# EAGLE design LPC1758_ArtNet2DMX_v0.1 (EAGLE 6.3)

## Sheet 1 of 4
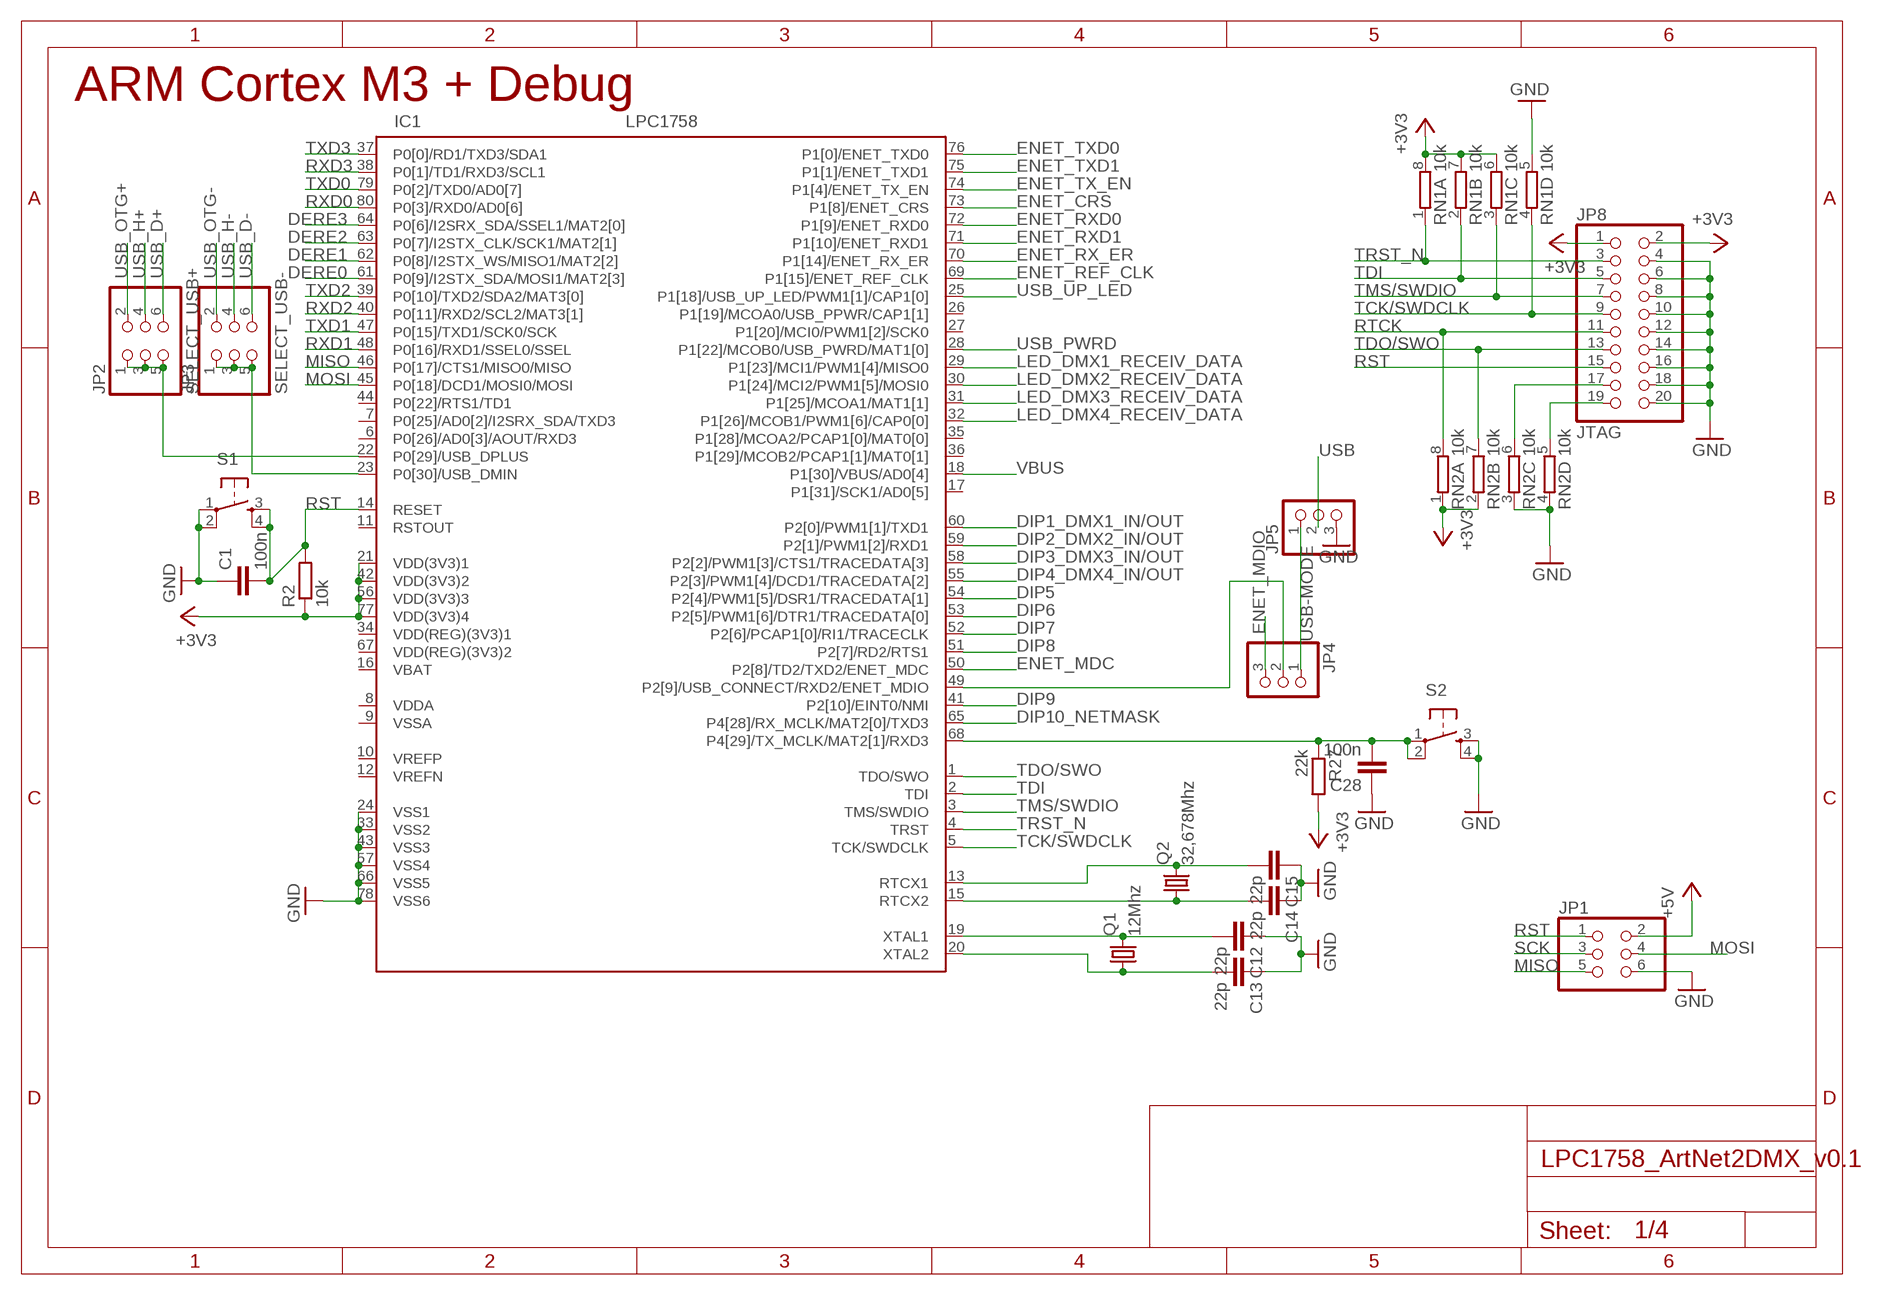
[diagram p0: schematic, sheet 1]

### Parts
C1  100n  C-EUC0805K  [C0805K]
C12  22p  C-EUC0805K  [C0805K]
C13  22p  C-EUC0805K  [C0805K]
C14  22p  C-EUC0805K  [C0805K]
C15  22p  C-EUC0805K  [C0805K]
C28  100n  C-EUC0805K  [C0805K]
IC1  LPC1758  [LQFP80-12X12]
JP1  PINHD-2X3_2.54-SMD  [2X03SMD]
JP2  SELECT_USB+  PINHD-2X3_2.54-SMD  [2X03SMD]
JP3  SELECT_USB-  PINHD-2X3_2.54-SMD  [2X03SMD]
JP4  PINHD-1X3_2.54-SMD  [1X03SMD]
JP5  PINHD-1X3_2.54-SMD  [1X03SMD]
JP8  JTAG  PINHD-2X10_2.54  [2X10]
Q1  12Mhz  CRYSTALSM49  [SM49]
Q2  32,678Mhz  CRYSTALSM49  [SM49]
R2  10k  R-EU_R0805  [R0805]
R27  22k  R-EU_R0805  [R0805]
RN1  10k  4R-NEXBS8V  [EXBS8V]
RN2  10k  4R-NEXBS8V  [EXBS8V]
S1  TASTER_93XX  [TASTER_93XX]
S2  TASTER_93XX  [TASTER_93XX]

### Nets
+3V3: IC1.21(VDD(3V3)1) IC1.42(VDD(3V3)2) IC1.56(VDD(3V3)3) IC1.77(VDD(3V3)4) JP8.1 JP8.2 R2.1 R27.2 RN1.6 RN1.7 RN1.8 RN2.1 RN2.2 ; also sheet 2,3,4
+5V: JP1.2 ; also sheet 3,4
BUTTON_RESERVE: C28.2 IC1.68(P4[29]/TX_MCLK/MAT2[1]/RXD3) R27.1 S2.1(P) S2.2(P1)
DERE0: IC1.61(P0[9]/I2STX_SDA/MOSI1/MAT2[3]) ; also sheet 3
DERE1: IC1.62(P0[8]/I2STX_WS/MISO1/MAT2[2]) ; also sheet 3
DERE2: IC1.63(P0[7]/I2STX_CLK/SCK1/MAT2[1]) ; also sheet 3
DERE3: IC1.64(P0[6]/I2SRX_SDA/SSEL1/MAT2[0]) ; also sheet 3
DIP1_DMX1_IN/OUT: IC1.60(P2[0]/PWM1[1]/TXD1) ; also sheet 3
DIP2_DMX2_IN/OUT: IC1.59(P2[1]/PWM1[2]/RXD1) ; also sheet 3
DIP3_DMX3_IN/OUT: IC1.58(P2[2]/PWM1[3]/CTS1/TRACEDATA[3]) ; also sheet 3
DIP4_DMX4_IN/OUT: IC1.55(P2[3]/PWM1[4]/DCD1/TRACEDATA[2]) ; also sheet 3
DIP5: IC1.54(P2[4]/PWM1[5]/DSR1/TRACEDATA[1]) ; also sheet 3
DIP6: IC1.53(P2[5]/PWM1[6]/DTR1/TRACEDATA[0]) ; also sheet 3
DIP7: IC1.52(P2[6]/PCAP1[0]/RI1/TRACECLK) ; also sheet 3
DIP8: IC1.51(P2[7]/RD2/RTS1) ; also sheet 3
DIP9: IC1.41(P2[10]/EINT0/NMI) ; also sheet 3
DIP10_NETMASK: IC1.65(P4[28]/RX_MCLK/MAT2[0]/TXD3) ; also sheet 3
ENET_CRS: IC1.73(P1[8]/ENET_CRS) ; also sheet 2
ENET_MDC: IC1.50(P2[8]/TD2/TXD2/ENET_MDC) ; also sheet 2
ENET_MDIO: JP4.3 ; also sheet 2
ENET_REF_CLK: IC1.69(P1[15]/ENET_REF_CLK) ; also sheet 2
ENET_RX_ER: IC1.70(P1[14]/ENET_RX_ER) ; also sheet 2
ENET_RXD0: IC1.72(P1[9]/ENET_RXD0) ; also sheet 2
ENET_RXD1: IC1.71(P1[10]/ENET_RXD1) ; also sheet 2
ENET_TX_EN: IC1.74(P1[4]/ENET_TX_EN) ; also sheet 2
ENET_TXD0: IC1.76(P1[0]/ENET_TXD0) ; also sheet 2
ENET_TXD1: IC1.75(P1[1]/ENET_TXD1) ; also sheet 2
GND: C1.1 C12.1 C13.1 C14.1 C15.1 C28.1 IC1.24(VSS1) IC1.33(VSS2) IC1.43(VSS3) IC1.57(VSS4) IC1.66(VSS5) IC1.78(VSS6) JP1.6 JP5.3 JP8.4 JP8.6 JP8.8 JP8.10 JP8.12 JP8.14 JP8.16 JP8.18 JP8.20 RN1.5 RN2.3 RN2.4 S1.1(P) S1.2(P1) S2.3(S) S2.4(S1) ; also sheet 2,3,4
LED_DMX1_RECEIV_DATA: IC1.29(P1[23]/MCI1/PWM1[4]/MISO0) ; also sheet 3
LED_DMX2_RECEIV_DATA: IC1.30(P1[24]/MCI2/PWM1[5]/MOSI0) ; also sheet 3
LED_DMX3_RECEIV_DATA: IC1.31(P1[25]/MCOA1/MAT1[1]) ; also sheet 3
LED_DMX4_RECEIV_DATA: IC1.32(P1[26]/MCOB1/PWM1[6]/CAP0[0]) ; also sheet 3
MISO: IC1.46(P0[17]/CTS1/MISO0/MISO) JP1.5
MOSI: IC1.45(P0[18]/DCD1/MOSI0/MOSI) JP1.4
N$12: C12.2 IC1.19(XTAL1) Q1.2
N$13: C13.2 IC1.20(XTAL2) Q1.1
N$16: C14.2 IC1.15(RTCX2) Q2.1
N$20: C15.2 IC1.13(RTCX1) Q2.2
N$22: IC1.22(P0[29]/USB_DPLUS) JP2.1 JP2.3 JP2.5
N$23: IC1.23(P0[30]/USB_DMIN) JP3.1 JP3.3 JP3.5
N$25: IC1.49(P2[9]/USB_CONNECT/RXD2/ENET_MDIO) JP4.2
N$42: JP8.19 RN2.5
N$43: JP8.17 RN2.6
RST: C1.2 IC1.14(RESET) JP1.1 JP8.15 R2.2 S1.3(S) S1.4(S1) ; also sheet 2
RTCK: JP8.11 RN2.8
RXD0: IC1.80(P0[3]/RXD0/AD0[6]) ; also sheet 3
RXD1: IC1.48(P0[16]/RXD1/SSEL0/SSEL) ; also sheet 3
RXD2: IC1.40(P0[11]/RXD2/SCL2/MAT3[1]) ; also sheet 3
RXD3: IC1.38(P0[1]/TD1/RXD3/SCL1) ; also sheet 3
SCK: JP1.3
TCK/SWDCLK: IC1.5(TCK/SWDCLK) JP8.9 RN1.4
TDI: IC1.2(TDI) JP8.5 RN1.2
TDO/SWO: IC1.1(TDO/SWO) JP8.13 RN2.7
TMS/SWDIO: IC1.3(TMS/SWDIO) JP8.7 RN1.3
TRST_N: IC1.4(TRST) JP8.3 RN1.1
TXD0: IC1.79(P0[2]/TXD0/AD0[7]) ; also sheet 3
TXD1: IC1.47(P0[15]/TXD1/SCK0/SCK) ; also sheet 3
TXD2: IC1.39(P0[10]/TXD2/SDA2/MAT3[0]) ; also sheet 3
TXD3: IC1.37(P0[0]/RD1/TXD3/SDA1) ; also sheet 3
USB: JP5.2 ; also sheet 4
USB-MODE: JP4.1 JP5.1
USB_D+: JP2.6 ; also sheet 4
USB_D-: JP3.6 ; also sheet 4
USB_H+: JP2.4
USB_H-: JP3.4
USB_OTG+: JP2.2
USB_OTG-: JP3.2
USB_PWRD: IC1.28(P1[22]/MCOB0/USB_PWRD/MAT1[0]) ; also sheet 4
USB_UP_LED: IC1.25(P1[18]/USB_UP_LED/PWM1[1]/CAP1[0]) ; also sheet 4
VBUS: IC1.18(P1[30]/VBUS/AD0[4]) ; also sheet 4
Unconnected: IC1.6(P0[26]/AD0[3]/AOUT/RXD3) IC1.7(P0[25]/AD0[2]/I2SRX_SDA/TXD3) IC1.10(VREFP) IC1.11(RSTOUT) IC1.12(VREFN) IC1.17(P1[31]/SCK1/AD0[5]) IC1.26(P1[19]/MCOA0/USB_PPWR/CAP1[1]) IC1.27(P1[20]/MCI0/PWM1[2]/SCK0) IC1.35(P1[28]/MCOA2/PCAP1[0]/MAT0[0]) IC1.36(P1[29]/MCOB2/PCAP1[1]/MAT0[1]) IC1.44(P0[22]/RTS1/TD1)

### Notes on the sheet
- ARM Cortex M3 + Debug

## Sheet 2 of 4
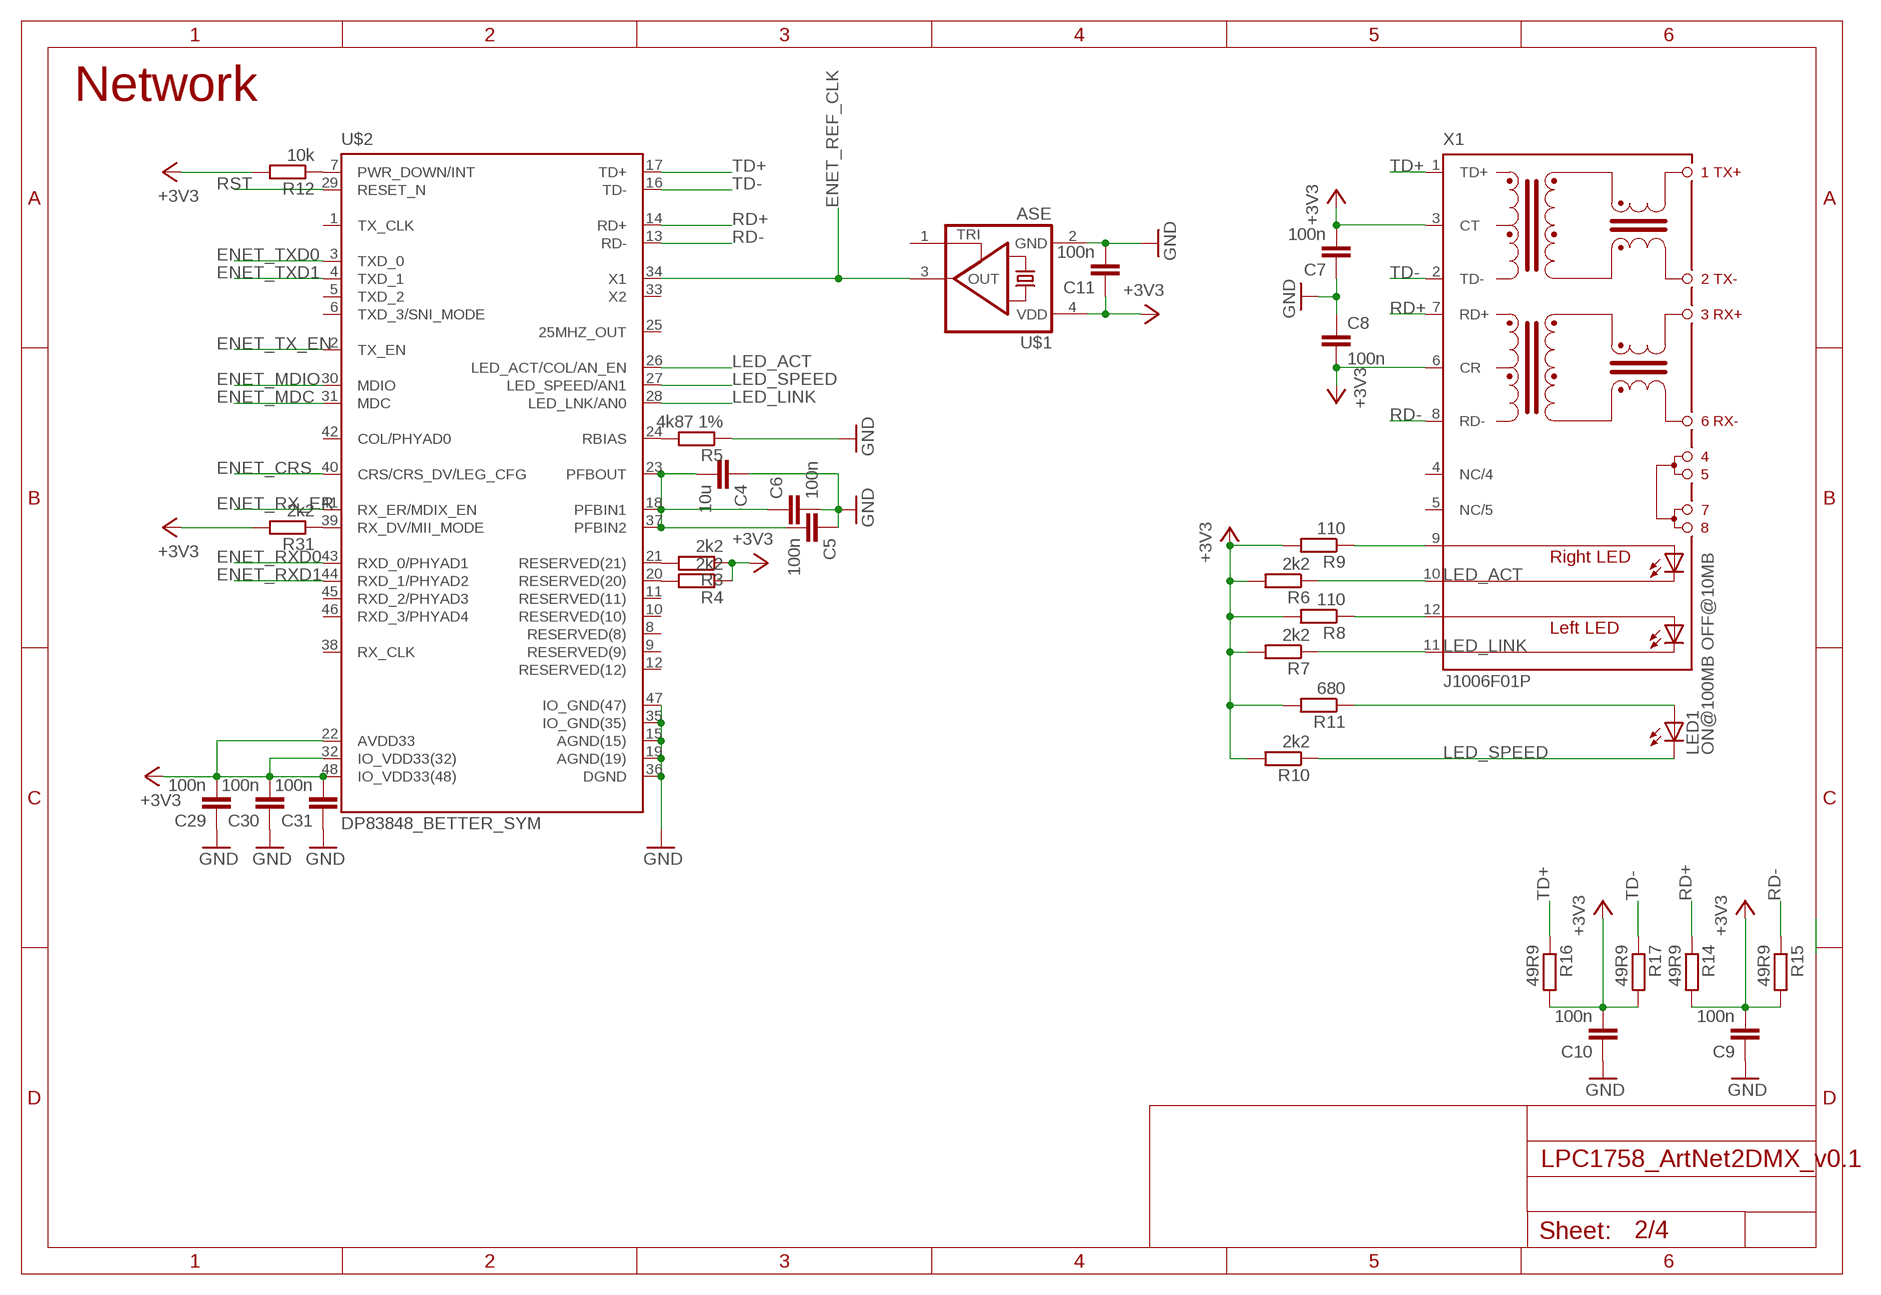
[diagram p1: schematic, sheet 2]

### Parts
C4  10u  C-EUC0805K  [C0805K]
C5  100n  C-EUC0805K  [C0805K]
C6  100n  C-EUC0805K  [C0805K]
C7  100n  C-EUC0805K  [C0805K]
C8  100n  C-EUC0805K  [C0805K]
C9  100n  C-EUC0805K  [C0805K]
C10  100n  C-EUC0805K  [C0805K]
C11  100n  C-EUC0805K  [C0805K]
C29  100n  C-EUC0805K  [C0805K]
C30  100n  C-EUC0805K  [C0805K]
C31  100n  C-EUC0805K  [C0805K]
LED1  ON@100MB OFF@10MB  LEDCHIP-LED0805  [CHIP-LED0805]
R3  2k2  R-EU_R0805  [R0805]
R4  2k2  R-EU_R0805  [R0805]
R5  4k87 1%  R-EU_R0805  [R0805]
R6  2k2  R-EU_R0805  [R0805]
R7  2k2  R-EU_R0805  [R0805]
R8  110  R-EU_R0805  [R0805]
R9  110  R-EU_R0805  [R0805]
R10  2k2  R-EU_R0805  [R0805]
R11  680  R-EU_R0805  [R0805]
R12  10k  R-EU_R0805  [R0805]
R14  49R9  R-EU_R0805  [R0805]
R15  49R9  R-EU_R0805  [R0805]
R16  49R9  R-EU_R0805  [R0805]
R17  49R9  R-EU_R0805  [R0805]
R31  2k2  R-EU_R0805  [R0805]
U$1  ASE  [ASE]
U$2  DP83848_BETTER_SYM  [LQFP48]
X1  J1006F01P  [J1]

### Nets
+3V3: C7.2 C8.2 C9.2 C10.2 C11.1 C29.2 C30.2 C31.2 R3.1 R4.1 R6.2 R7.2 R8.2 R9.2 R10.2 R11.2 R12.2 R14.2 R15.2 R16.2 R17.2 R31.2 U$1.4(VDD) U$2.22(AVDD33) U$2.32(IO_VDD33(32)) U$2.48(IO_VDD33(48)) X1.3(CT) X1.6(CR) ; also sheet 1,3,4
ENET_CRS: U$2.40(CRS/CRS_DV/LEG_CFG) ; also sheet 1
ENET_MDC: U$2.31(MDC) ; also sheet 1
ENET_MDIO: U$2.30(MDIO) ; also sheet 1
ENET_REF_CLK: U$1.3(OUT) U$2.34(X1) ; also sheet 1
ENET_RX_ER: U$2.41(RX_ER/MDIX_EN) ; also sheet 1
ENET_RXD0: U$2.43(RXD_0/PHYAD1) ; also sheet 1
ENET_RXD1: U$2.44(RXD_1/PHYAD2) ; also sheet 1
ENET_TX_EN: U$2.2(TX_EN) ; also sheet 1
ENET_TXD0: U$2.3(TXD_0) ; also sheet 1
ENET_TXD1: U$2.4(TXD_1) ; also sheet 1
GND: C4.1 C5.1 C6.2 C7.1 C8.1 C9.1 C10.1 C11.2 C29.1 C30.1 C31.1 R5.1 U$1.2(GND) U$2.15(AGND(15)) U$2.19(AGND(19)) U$2.35(IO_GND(35)) U$2.36(DGND) U$2.47(IO_GND(47)) ; also sheet 1,3,4
LED_ACT: R6.1 U$2.26(LED_ACT/COL/AN_EN) X1.10(C-R)
LED_LINK: R7.1 U$2.28(LED_LNK/AN0) X1.11(C-L)
LED_SPEED: LED1.C R10.1 U$2.27(LED_SPEED/AN1)
N$4: R8.1 X1.12(A-L)
N$8: R9.1 X1.9(A-R)
N$9: LED1.A R11.1
N$10: R12.1 U$2.7(PWR_DOWN/INT)
N$14: R3.2 U$2.21(RESERVED(21))
N$15: R4.2 U$2.20(RESERVED(20))
N$17: C4.2 C5.2 C6.1 U$2.18(PFBIN1) U$2.23(PFBOUT) U$2.37(PFBIN2)
N$18: R5.2 U$2.24(RBIAS)
N$19: R31.1 U$2.39(RX_DV/MII_MODE)
RD+: R14.1 U$2.14(RD+) X1.7(RD+)
RD-: R15.1 U$2.13(RD-) X1.8(RD-)
RST: U$2.29(RESET_N) ; also sheet 1
TD+: R16.1 U$2.17(TD+) X1.1(TD+)
TD-: R17.1 U$2.16(TD-) X1.2(TD-)
Unconnected: U$1.1(TRI) U$2.1(TX_CLK) U$2.5(TXD_2) U$2.6(TXD_3/SNI_MODE) U$2.8(RESERVED(8)) U$2.9(RESERVED(9)) U$2.10(RESERVED(10)) U$2.11(RESERVED(11)) U$2.12(RESERVED(12)) U$2.25(25MHZ_OUT) U$2.33(X2) U$2.38(RX_CLK) U$2.42(COL/PHYAD0) U$2.45(RXD_2/PHYAD3) U$2.46(RXD_3/PHYAD4) X1.4(NC/4) X1.5(NC/5)

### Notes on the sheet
- Network

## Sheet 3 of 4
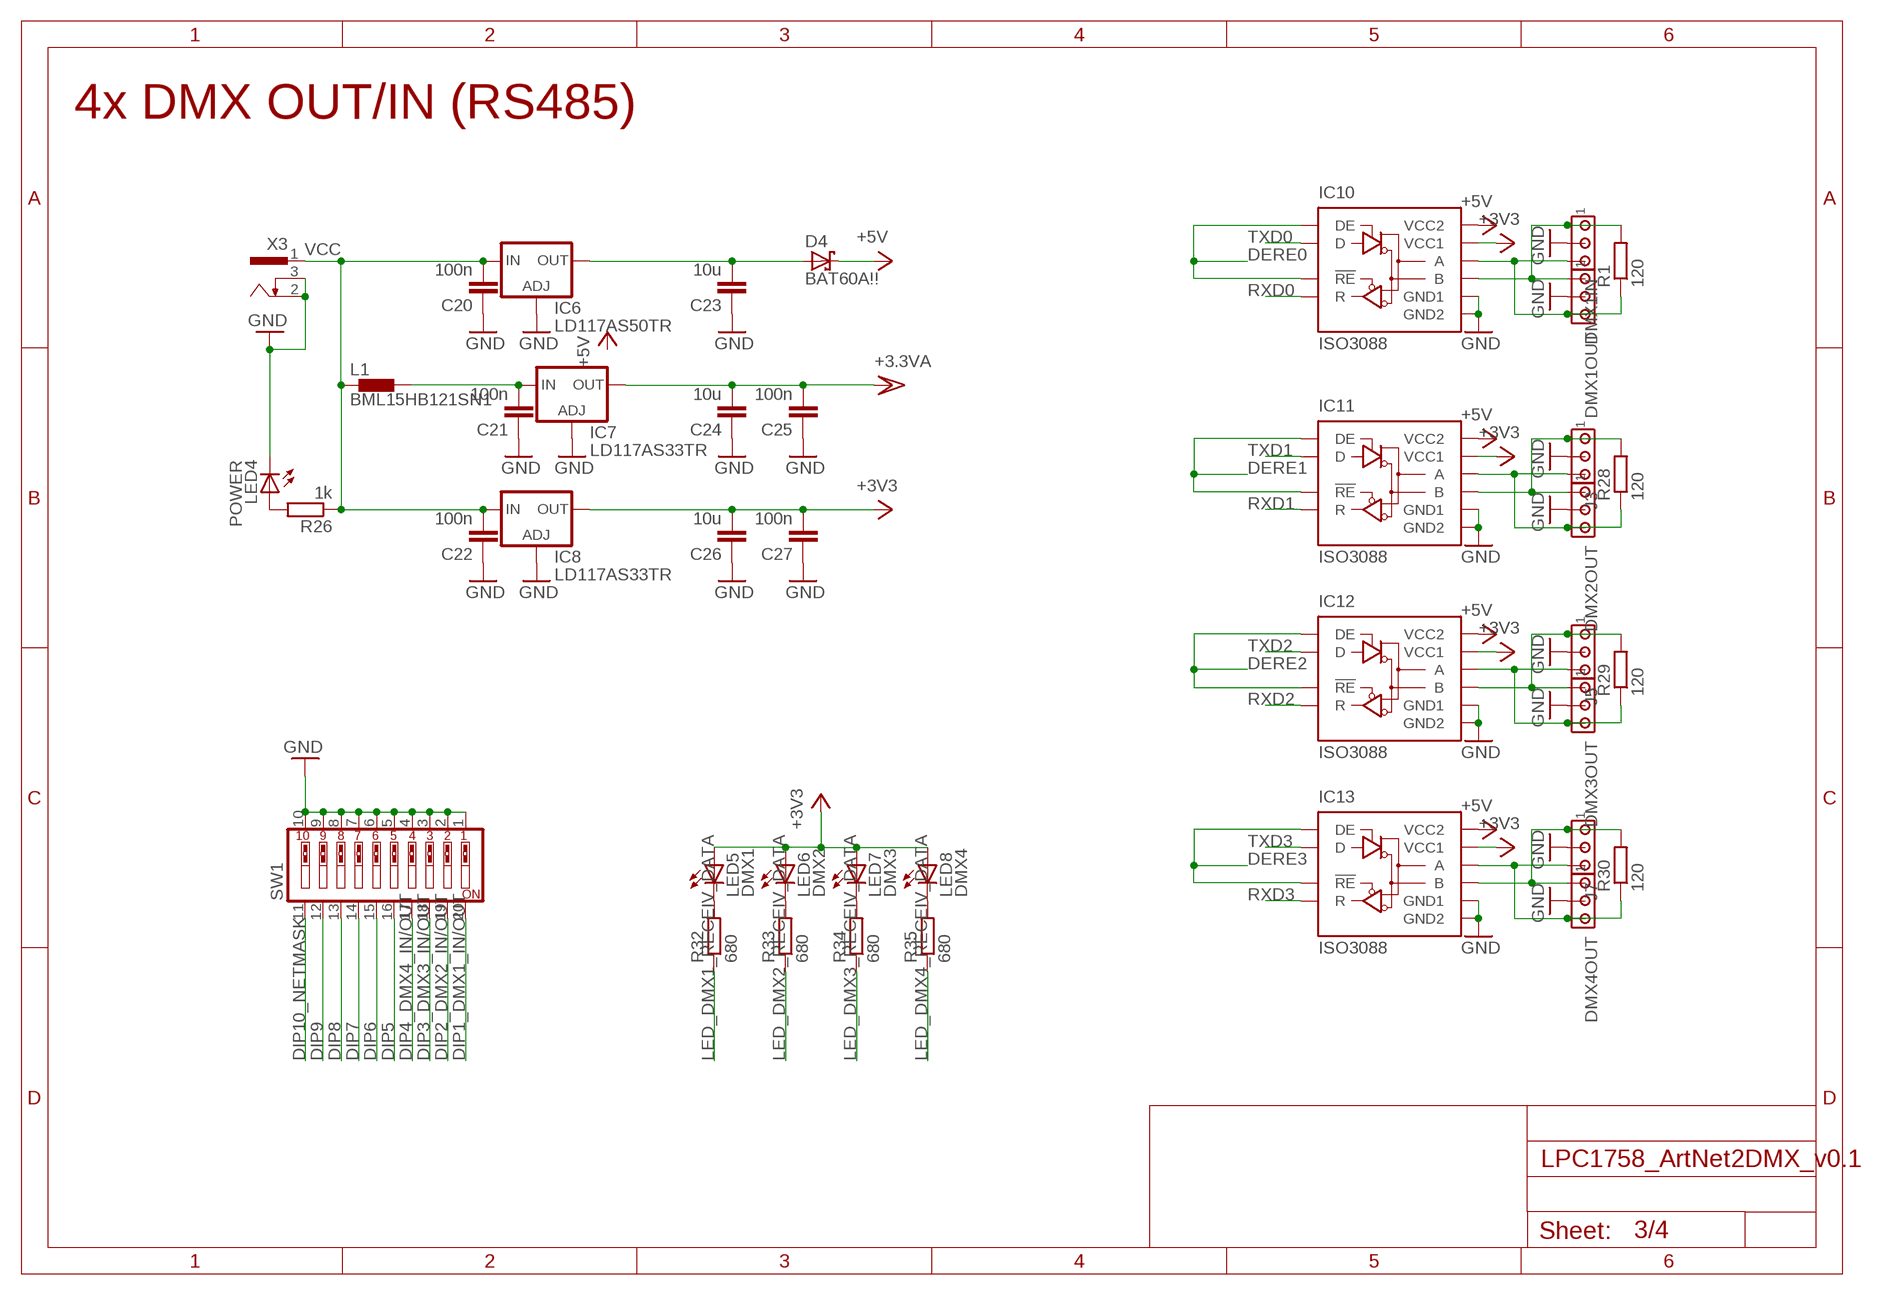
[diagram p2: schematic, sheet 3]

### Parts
C20  100n  C-EUC0805K  [C0805K]
C21  100n  C-EUC0805K  [C0805K]
C22  100n  C-EUC0805K  [C0805K]
C23  10u  C-EUC0805K  [C0805K]
C24  10u  C-EUC0805K  [C0805K]
C25  100n  C-EUC0805K  [C0805K]
C26  10u  C-EUC0805K  [C0805K]
C27  100n  C-EUC0805K  [C0805K]
D4  BAT60A!!  BAT54  [SOT23]
DMX1IN  MTA03-100  [10X03MTA]
DMX1OUT  MTA03-100  [10X03MTA]
DMX2OUT  MTA03-100  [10X03MTA]
DMX3OUT  MTA03-100  [10X03MTA]
DMX4OUT  MTA03-100  [10X03MTA]
IC6  LD117AS50TR  [SOT223]
IC7  LD117AS33TR  [SOT223]
IC8  LD117AS33TR  [SOT223]
IC10  ISO3088  [SO16]
IC11  ISO3088  [SO16]
IC12  ISO3088  [SO16]
IC13  ISO3088  [SO16]
J3  MTA03-100  [10X03MTA]
J5  MTA03-100  [10X03MTA]
J7  MTA03-100  [10X03MTA]
L1  BML15HB121SN1  [0402]
LED4  POWER  LEDCHIP-LED0805  [CHIP-LED0805]
LED5  DMX1  LEDCHIP-LED0805  [CHIP-LED0805]
LED6  DMX2  LEDCHIP-LED0805  [CHIP-LED0805]
LED7  DMX3  LEDCHIP-LED0805  [CHIP-LED0805]
LED8  DMX4  LEDCHIP-LED0805  [CHIP-LED0805]
R1  120  R-EU_R0805  [R0805]
R26  1k  R-EU_R0805  [R0805]
R28  120  R-EU_R0805  [R0805]
R29  120  R-EU_R0805  [R0805]
R30  120  R-EU_R0805  [R0805]
R32  680  R-EU_R0805  [R0805]
R33  680  R-EU_R0805  [R0805]
R34  680  R-EU_R0805  [R0805]
R35  680  R-EU_R0805  [R0805]
SW1  SW_DIP-10  [EDG-10]
X3  733980-62  [733980-62]

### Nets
+3.3VA: C24.2 C25.2 IC7.4(OUT)
+3V3: C26.2 C27.2 IC8.4(OUT) IC10.1(VCC1) IC11.1(VCC1) IC12.1(VCC1) IC13.1(VCC1) LED5.A LED6.A LED7.A LED8.A ; also sheet 1,2,4
+5V: D4.3(C) IC10.16(VCC2) IC11.16(VCC2) IC12.16(VCC2) IC13.16(VCC2) ; also sheet 1,4
DERE0: IC10.4(!RE) IC10.5(DE) ; also sheet 1
DERE1: IC11.4(!RE) IC11.5(DE) ; also sheet 1
DERE2: IC12.4(!RE) IC12.5(DE) ; also sheet 1
DERE3: IC13.4(!RE) IC13.5(DE) ; also sheet 1
DIP1_DMX1_IN/OUT: SW1.20 ; also sheet 1
DIP2_DMX2_IN/OUT: SW1.19 ; also sheet 1
DIP3_DMX3_IN/OUT: SW1.18 ; also sheet 1
DIP4_DMX4_IN/OUT: SW1.17 ; also sheet 1
DIP5: SW1.16 ; also sheet 1
DIP6: SW1.15 ; also sheet 1
DIP7: SW1.14 ; also sheet 1
DIP8: SW1.13 ; also sheet 1
DIP9: SW1.12 ; also sheet 1
DIP10_NETMASK: SW1.11 ; also sheet 1
GND: C20.1 C21.1 C22.1 C23.1 C24.1 C25.1 C26.1 C27.1 DMX1IN.2 DMX1OUT.2 DMX2OUT.2 DMX3OUT.2 DMX4OUT.2 IC6.1(ADJ) IC7.1(ADJ) IC8.1(ADJ) IC10.2(GND1) IC10.7(GND1) IC10.8(GND1) IC10.9(GND2) IC10.10(GND2) IC10.15(GND2) IC11.2(GND1) IC11.7(GND1) IC11.8(GND1) IC11.9(GND2) IC11.10(GND2) IC11.15(GND2) IC12.2(GND1) IC12.7(GND1) IC12.8(GND1) IC12.9(GND2) IC12.10(GND2) IC12.15(GND2) IC13.2(GND1) IC13.7(GND1) IC13.8(GND1) IC13.9(GND2) IC13.10(GND2) IC13.15(GND2) J3.2 J5.2 J7.2 LED4.C SW1.1 SW1.2 SW1.3 SW1.4 SW1.5 SW1.6 SW1.7 SW1.8 SW1.9 SW1.10 X3.2 X3.3 ; also sheet 1,2,4
LED_DMX1_RECEIV_DATA: R32.1 ; also sheet 1
LED_DMX2_RECEIV_DATA: R33.1 ; also sheet 1
LED_DMX3_RECEIV_DATA: R34.1 ; also sheet 1
LED_DMX4_RECEIV_DATA: R35.1 ; also sheet 1
N$1: DMX1IN.3 DMX1OUT.3 IC10.12(A) R1.1
N$2: DMX1IN.1 DMX1OUT.1 IC10.13(B) R1.2
N$5: LED5.C R32.2
N$6: LED6.C R33.2
N$11: C21.2 IC7.3(IN) L1.2
N$32: LED4.A R26.2
N$35: C23.2 D4.1(A) IC6.4(OUT)
N$36: DMX2OUT.3 IC11.12(A) J3.3 R28.1
N$37: DMX2OUT.1 IC11.13(B) J3.1 R28.2
N$38: DMX3OUT.3 IC12.12(A) J5.3 R29.1
N$39: DMX3OUT.1 IC12.13(B) J5.1 R29.2
N$40: DMX4OUT.3 IC13.12(A) J7.3 R30.1
N$41: DMX4OUT.1 IC13.13(B) J7.1 R30.2
N$44: LED7.C R34.2
N$45: LED8.C R35.2
RXD0: IC10.3(R) ; also sheet 1
RXD1: IC11.3(R) ; also sheet 1
RXD2: IC12.3(R) ; also sheet 1
RXD3: IC13.3(R) ; also sheet 1
TXD0: IC10.6(D) ; also sheet 1
TXD1: IC11.6(D) ; also sheet 1
TXD2: IC12.6(D) ; also sheet 1
TXD3: IC13.6(D) ; also sheet 1
VCC: C20.2 C22.2 IC6.3(IN) IC8.3(IN) L1.1 R26.1 X3.1 ; also sheet 4

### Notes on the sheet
- 4x DMX OUT/IN (RS485)

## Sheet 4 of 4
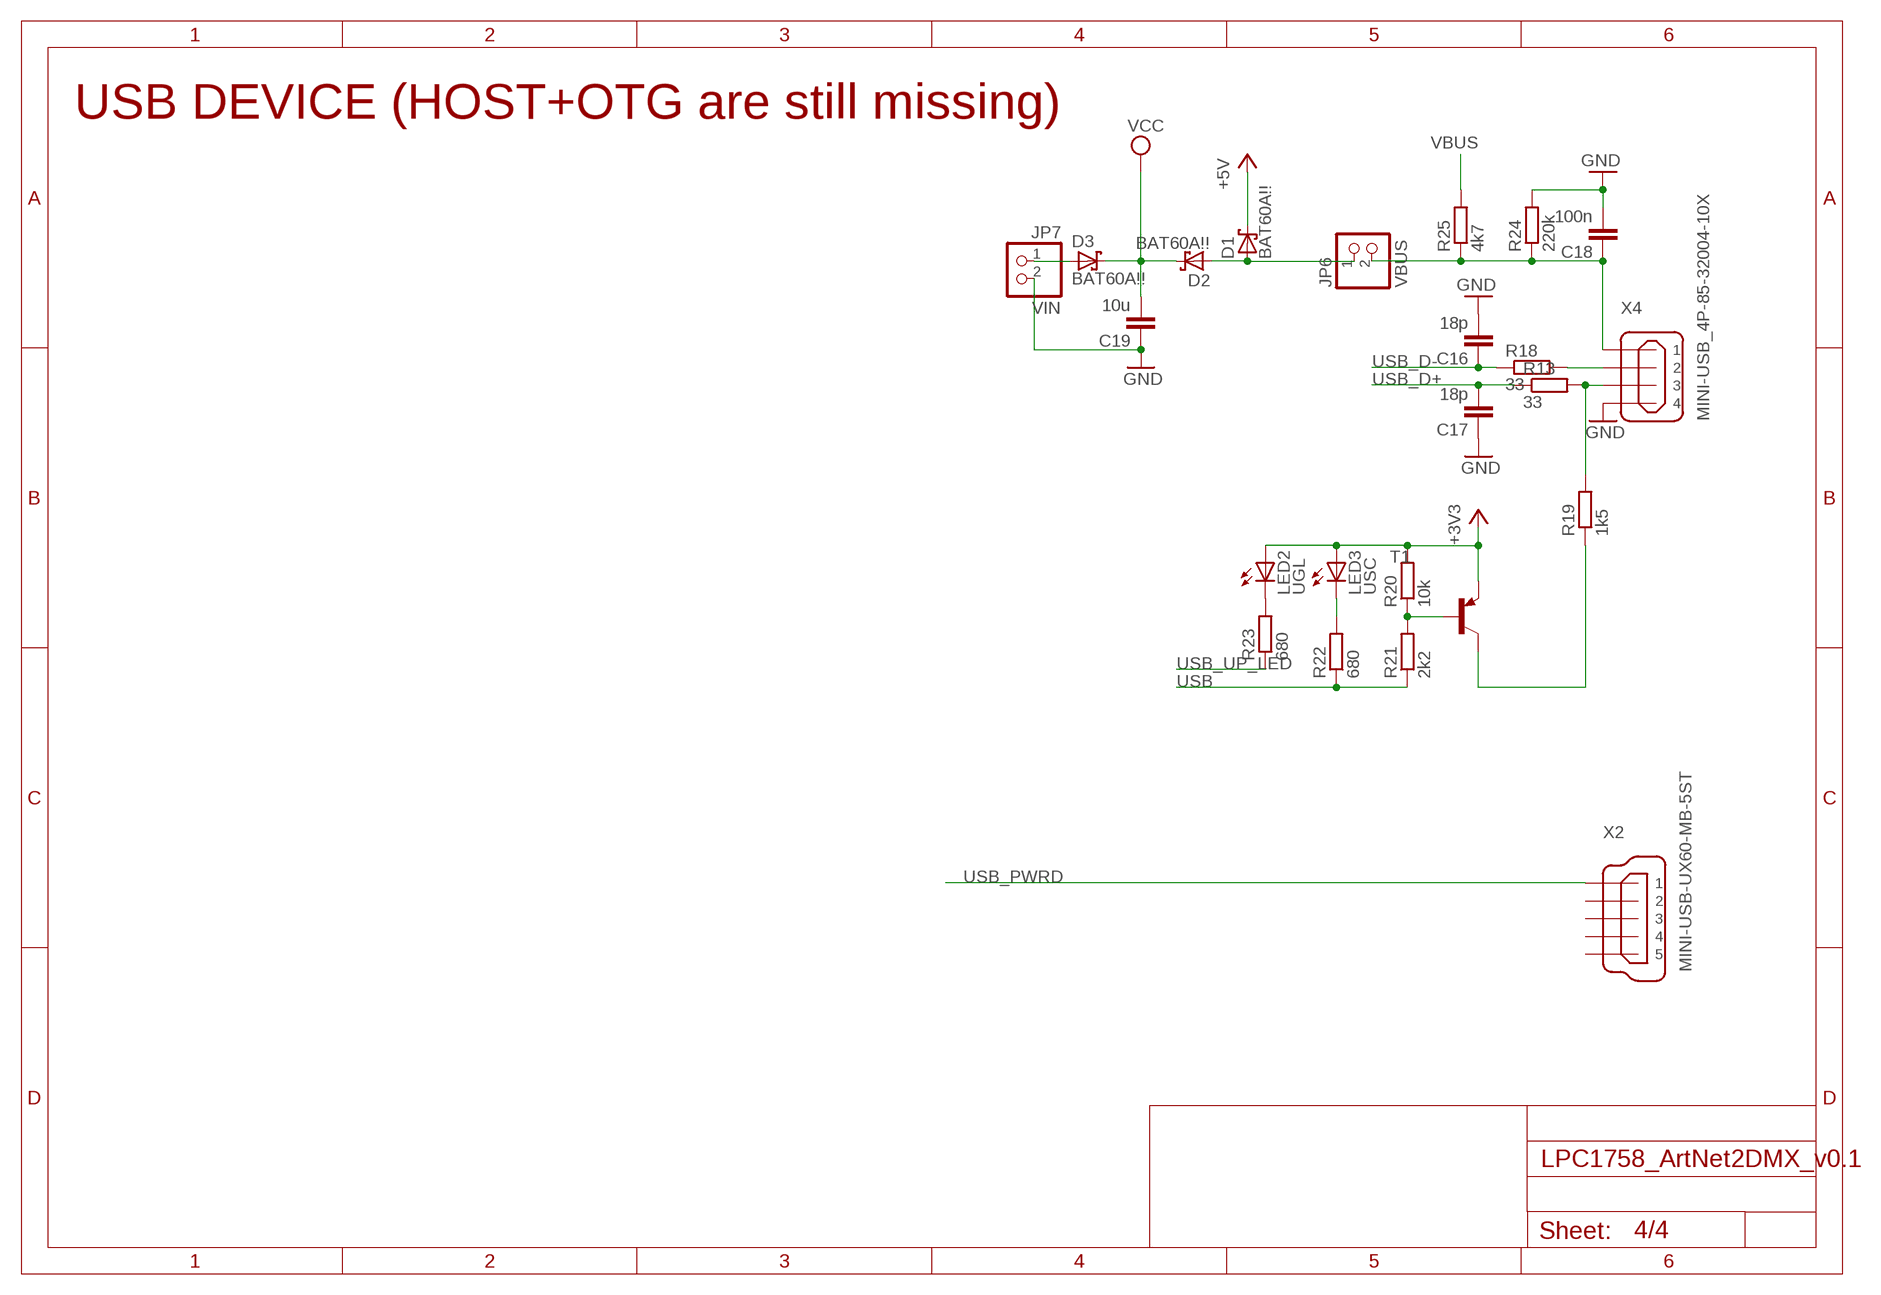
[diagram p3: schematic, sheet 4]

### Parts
C16  18p  C-EUC0805K  [C0805K]
C17  18p  C-EUC0805K  [C0805K]
C18  100n  C-EUC0805K  [C0805K]
C19  10u  C-EUC0805K  [C0805K]
D1  BAT60A!!  BAT54  [SOT23]
D2  BAT60A!!  BAT54  [SOT23]
D3  BAT60A!!  BAT54  [SOT23]
JP6  VBUS  PINHD-1X2_2.54-SMD  [1X02SMD]
JP7  VIN  PINHD-1X2_2.54-SMD  [1X02SMD]
LED2  UGL  LEDCHIP-LED0805  [CHIP-LED0805]
LED3  USC  LEDCHIP-LED0805  [CHIP-LED0805]
R13  33  R-EU_R0805  [R0805]
R18  33  R-EU_R0805  [R0805]
R19  1k5  R-EU_R0805  [R0805]
R20  10k  R-EU_R0805  [R0805]
R21  2k2  R-EU_R0805  [R0805]
R22  680  R-EU_R0805  [R0805]
R23  680  R-EU_R0805  [R0805]
R24  220k  R-EU_R0805  [R0805]
R25  4k7  R-EU_R0805  [R0805]
T1  BC857B-PNP-SOT23-BEC  [SOT23-BEC]
X2  MINI-USB-UX60-MB-5ST  [UX60-MB-5ST]
X4  MINI-USB_4P-85-32004-10X  [85-32004-10X]

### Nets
+3V3: LED2.A LED3.A R20.2 T1.E ; also sheet 1,2,3
+5V: D1.3(C) ; also sheet 1,3
GND: C16.2 C17.1 C18.2 C19.1 JP7.2 R24.2 X4.4 ; also sheet 1,2,3
N$21: R18.2 X4.2
N$24: R13.2 R19.2 X4.3
N$26: R19.1 T1.C
N$27: LED2.C R23.2
N$28: R20.1 R21.2 T1.B
N$29: LED3.C R22.2
N$30: C18.1 JP6.2 R24.1 R25.1 X4.1
N$31: D1.1(A) D2.1(A) JP6.1
N$33: D3.1(A) JP7.1
USB: R21.1 R22.1 ; also sheet 1
USB_D+: C17.2 R13.1 ; also sheet 1
USB_D-: C16.1 R18.1 ; also sheet 1
USB_PWRD: X2.1 ; also sheet 1
USB_UP_LED: R23.1 ; also sheet 1
VBUS: R25.2 ; also sheet 1
VCC: C19.2 D2.3(C) D3.3(C) ; also sheet 3
Unconnected: X2.2 X2.3 X2.4 X2.5

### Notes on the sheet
- USB DEVICE (HOST+OTG are still missing)

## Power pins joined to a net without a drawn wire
VBAT: IC1.16(VBAT)
VDD(REG)(3V3)1: IC1.34(VDD(REG)(3V3)1)
VDD(REG)(3V3)2: IC1.67(VDD(REG)(3V3)2)
VDDA: IC1.8(VDDA)
VSSA: IC1.9(VSSA)

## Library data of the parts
C1 C4-C31 = resistor:C-EU: CAPACITOR, European symbol
D1-D4 = diode:BAT54: Schottky Diodes
DMX1IN DMX1OUT DMX2OUT DMX3OUT DMX4OUT J3 J5 J7 = con-amp:MTA03-100: AMP connector
IC1 = lpc1xxx-v6:LPC1758: LPC1758 100 MHz 32-bit ARM Cortex-M3 based microcontroller featuring a high level of integration and low power consumption. 512 kB Flash, 64 kB SRAM, USB Device/Host/OTG, 2 CAN, DAC, Ethernet MarcVl - Datasheet available on www.nxp.com
IC6-IC8 = v-reg:LD117A?*: Low drop fixed and adjustable positive voltage regulators 1 A Source: http://www.st.com/stonline/products/literature/ds/7194/ld1117axx.pdf
IC10-IC13 = iso308x_RS485:ISO3088
JP1-JP3 = pinhead-1:PINHD-2X3: PIN HEADER
JP4 JP5 = pinhead-1:PINHD-1X3: PIN HEADER
JP6 JP7 = pinhead-1:PINHD-1X2: PIN HEADER
JP8 = pinhead-1:PINHD-2X10: PIN HEADER
L1 = inductors:BML15H: EMIFIL (R) Chip Ferrite Bead for GHz Noise
LED1-LED8 = led:LED: LED
Q1 Q2 = crystal:CRYSTAL: CRYSTAL; OC_FARNELL: unknown; OC_NEWARK: unknown
R1-R35 = resistor:R-EU_: RESISTOR, European symbol
RN1 RN2 = resistor-dil:4R-N: Array Chip Resistor Source: RS Component / Phycomp; OC_FARNELL: unknown; OC_NEWARK: unknown
S1 S2 = uwegw:TASTER_93XX: OMRON SWITCH
SW1 = special:SW_DIP-10: DIP SWITCH
T1 = transistor:*-PNP-: PNP Transistror
U$1 = crystal:ASE: 3.3Vdc CMOS SMD CRYSTAL CLOCK OSCILLATOR SOurce: www.abracon.com; OC_FARNELL: unknown; OC_NEWARK: unknown
U$2 = national-semiconductor:DP83848_BETTER_SYM
X1 = con-pulse:J1006F01P: PULSEJACK (TM) 1x1 Tab-UP RJ45 10/100 Base-TX RJ45 1x1 Tab-UP with LEDs 8-pin (J1 series) and 6-pin (JP series) integrated magnetics connector, designed to support applications, such as ADSL modems, LAN-on-Motherboard, and Hub and Switches. Source: www.pulseeng.com .. PulseJack-J402.pdf; OC_FARNELL: unknown; OC_NEWARK: unknown
X2 = con-hirose:MINI-USB-: MINI USB Connector Source: http://www.hirose.co.jp/cataloge_hp/e24000019.pdf; OC_FARNELL: unknown; OC_NEWARK: unknown
X3 = con-conrad:73398?: FEMALE PRINT CONNECTOR Niedervolt-Steckverbinder Distributor Conrad
X4 = con-cypressindustries:MINI-USB_4P-: MINI USB 4 Pol. Source: www.cypressindustries.com; OC_FARNELL: unknown; OC_NEWARK: unknown

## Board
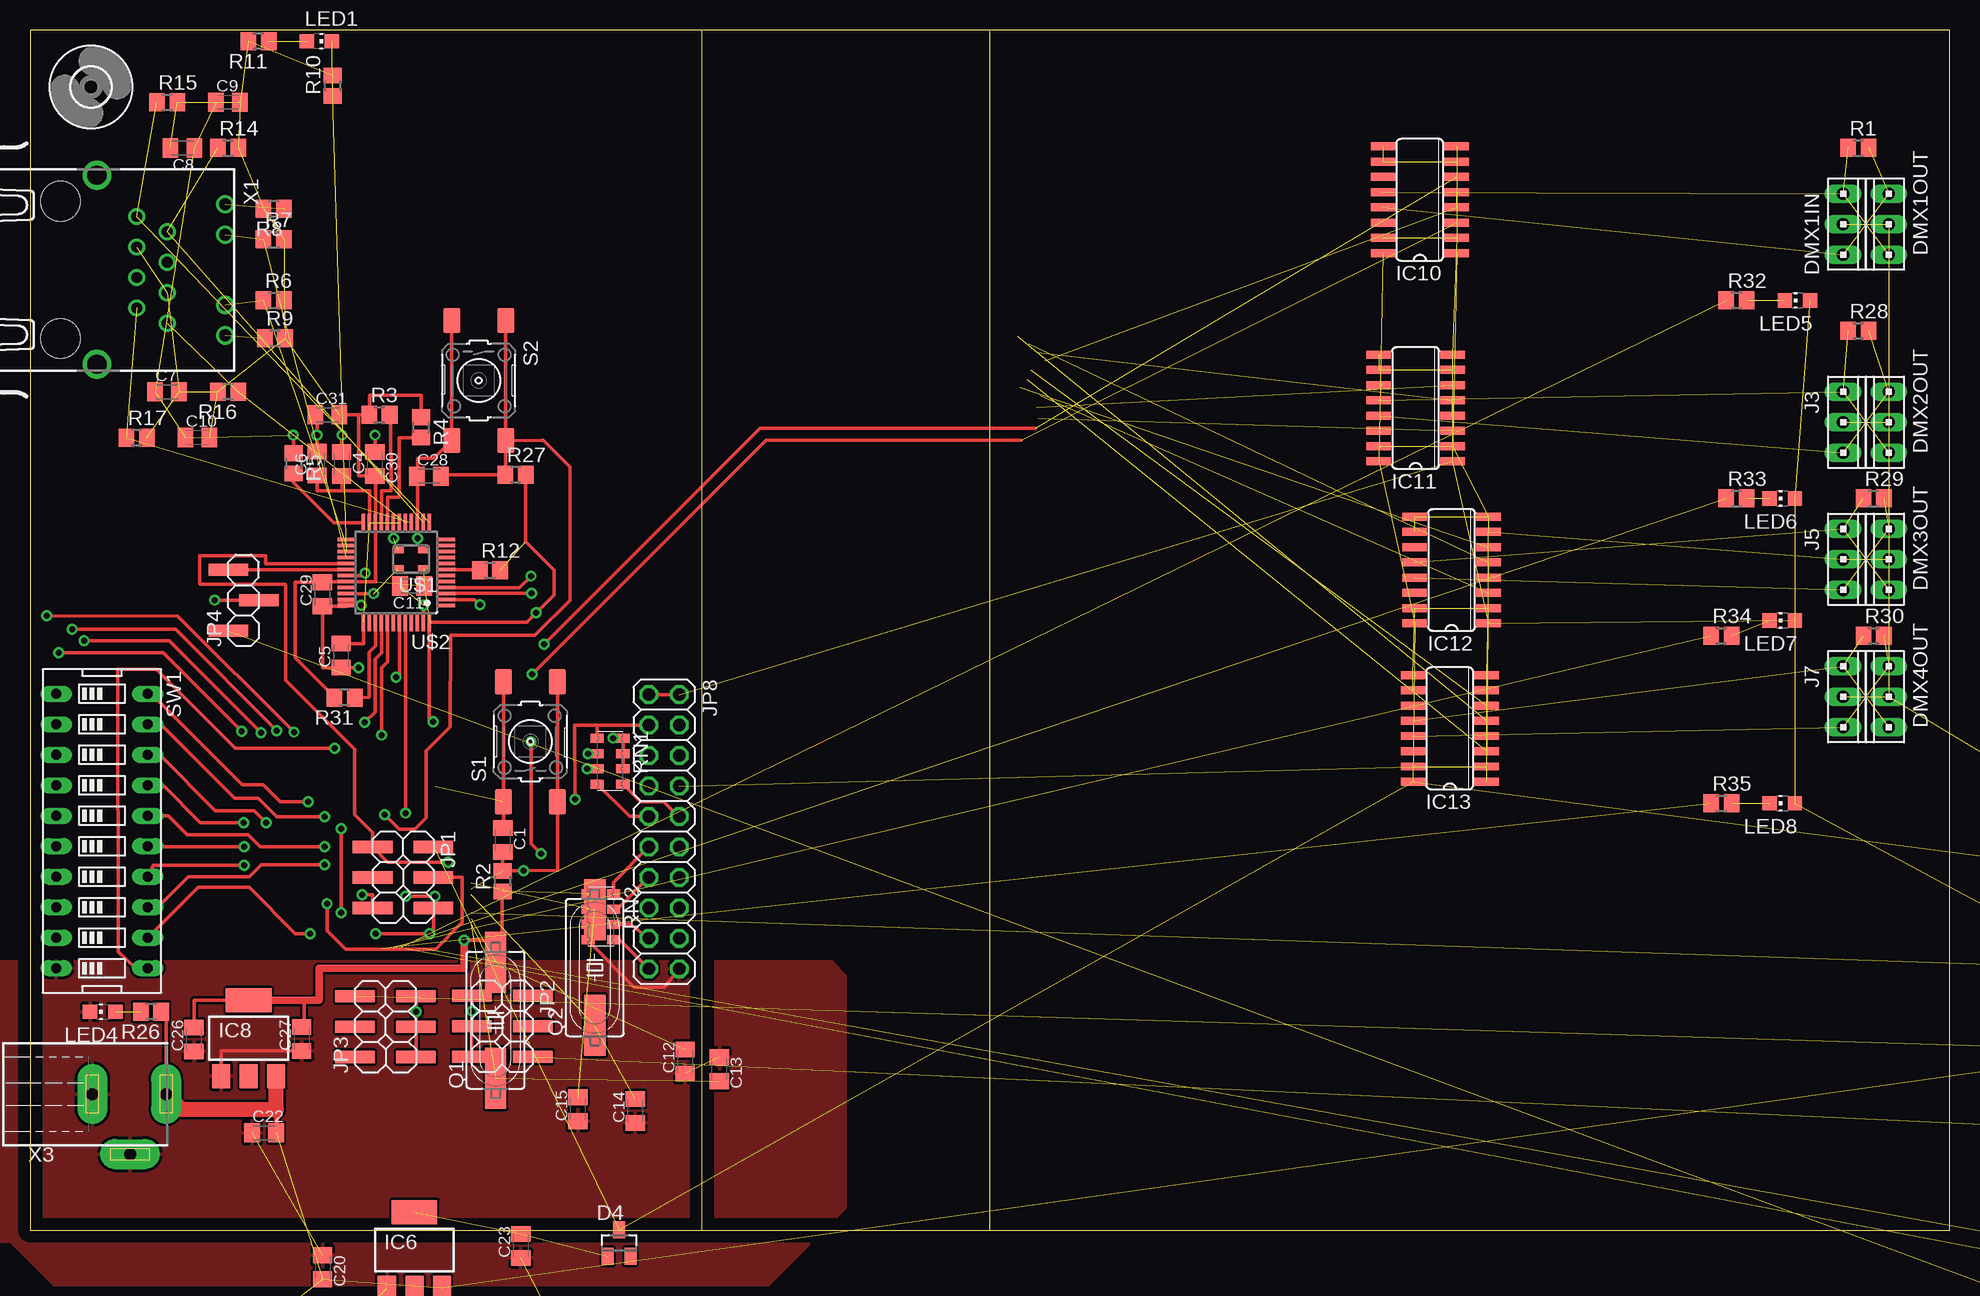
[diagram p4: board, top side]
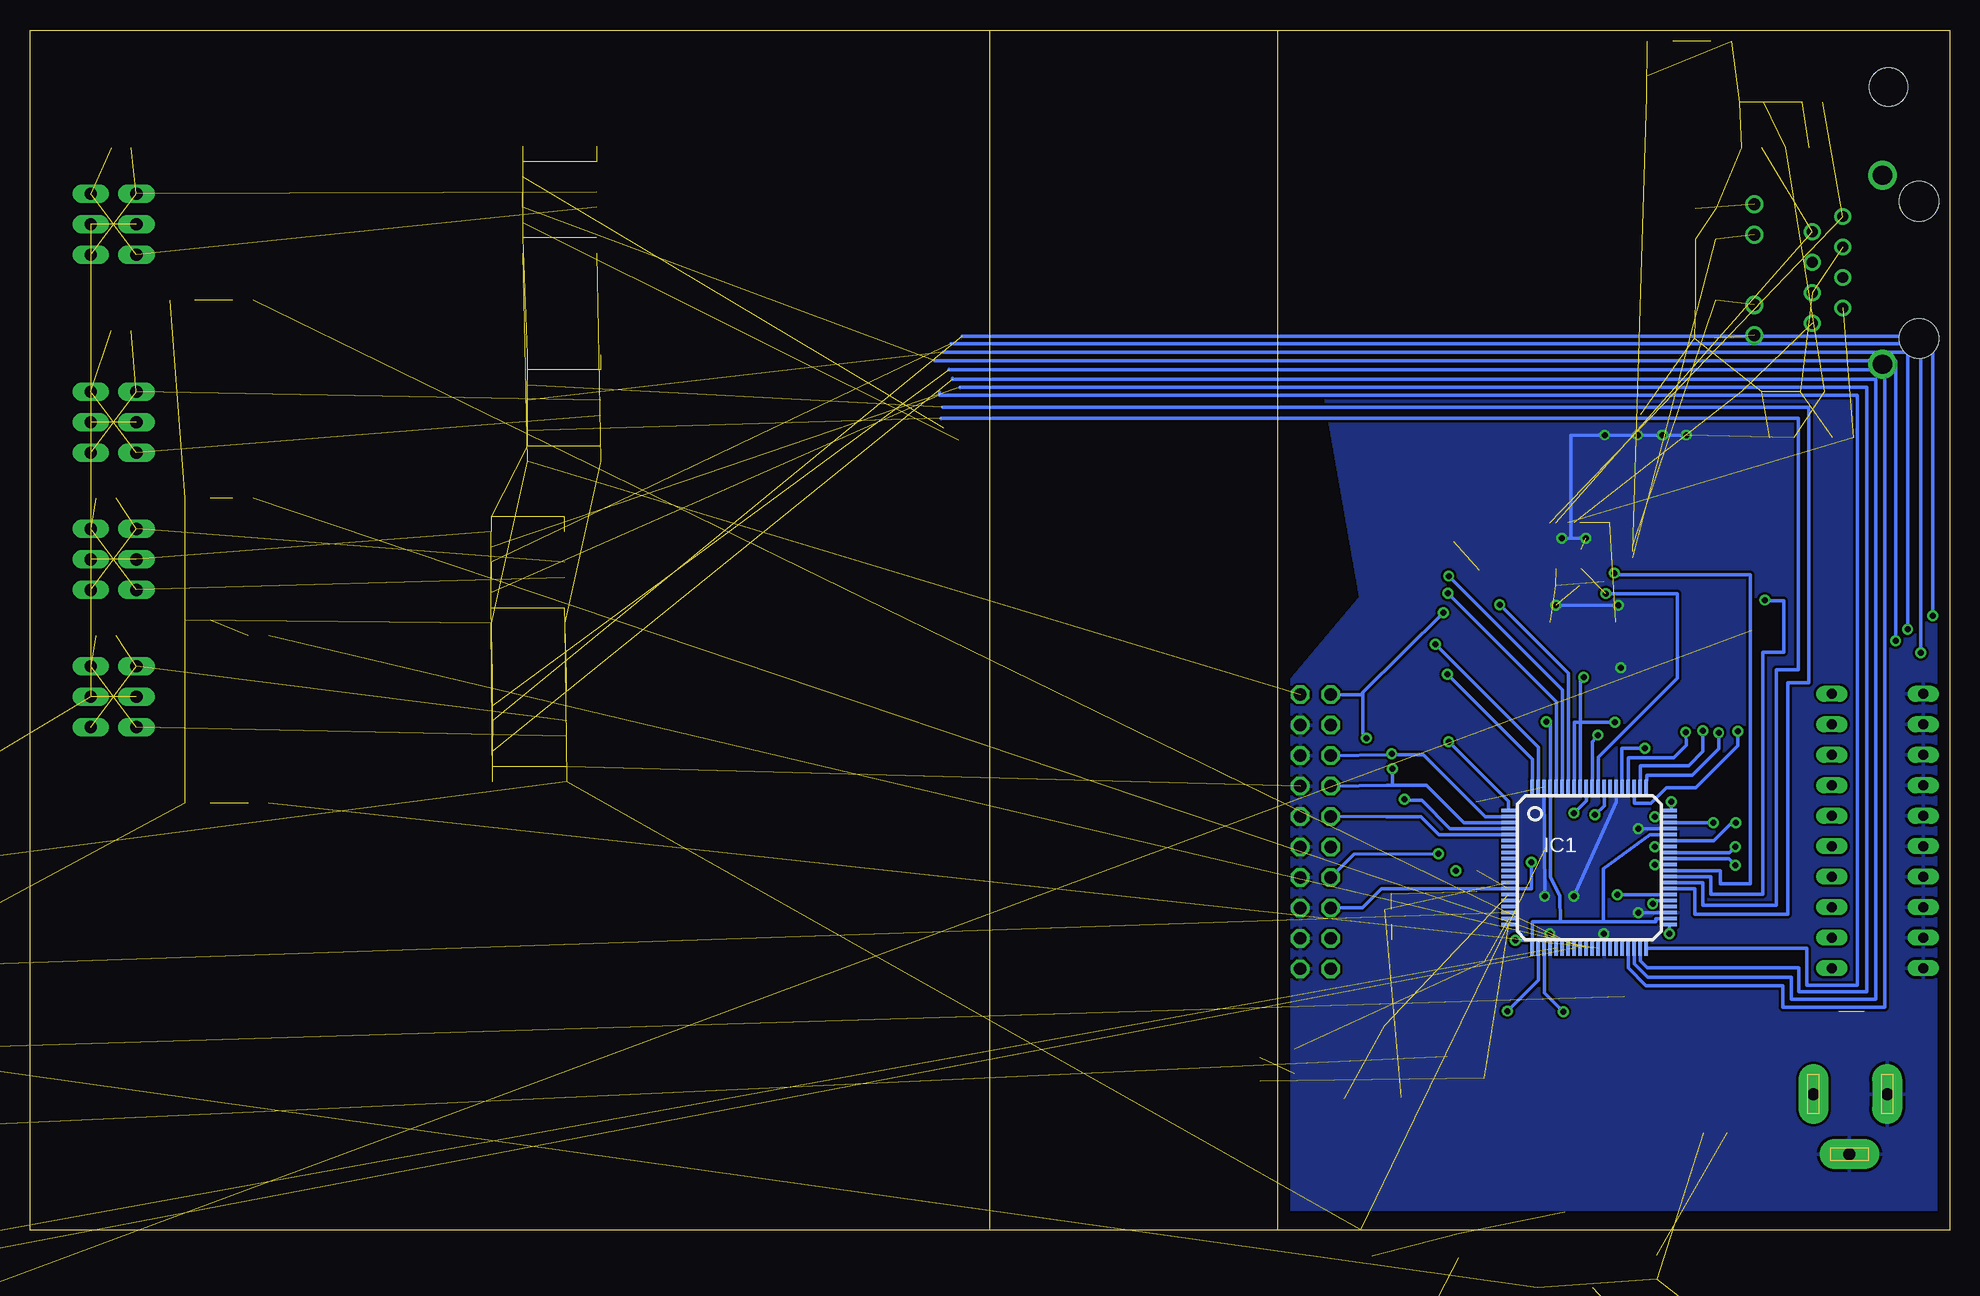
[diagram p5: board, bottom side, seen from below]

Size 160 x 100 mm. Coordinates in mm from the lower left corner, seen from the top.
Outline: 56,0 0,0 0,100 56,100
Outline: 56,0 80,0
Outline: 80,0 160,0 160,100 80,100
Outline: 80,100 56,100
Outline: 80,0 80,100
Outline: 56,0 56,100
Copper layers (1*16): Top 0.035mm / dielectric 1.5mm / Bottom 0.035mm
Design rules "default": minimum track width 10mil, minimum drill 24mil, track to track 8mil, track to pad 8mil, pad to pad 8mil, via to via 8mil, smd to smd 8mil, copper to edge 40mil, drill to drill 8mil, minimum pad ring 10mil, minimum via ring 8mil, stop-mask expansion 4mil, vias tented up to drill 0mil, thermal gap 10mil

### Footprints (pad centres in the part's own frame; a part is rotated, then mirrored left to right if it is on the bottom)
C0805K = smd 1.3 x 1.6: 1 -1,0; 2 1,0
SOT23 = smd 1 x 1.4: 1 -0.95,-1.1; 2 0.95,-1.1; 3 0,1.1
10X03MTA = drill 1.016 long: 1 2.54,0; 2 0,0; 3 -2.54,0
LQFP80-12X12 = smd 1.2 x 0.3: 1 -6.725,4.75; 2 -6.725,4.25; 3 -6.725,3.75; 4 -6.725,3.25; 5 -6.725,2.75; 6 -6.725,2.25; 7 -6.725,1.75; 8 -6.725,1.25; 9 -6.725,0.75; 10 -6.725,0.25; 11 -6.725,-0.25; 12 -6.725,-0.75; 13 -6.725,-1.25; 14 -6.725,-1.75; 15 -6.725,-2.25; 16 -6.725,-2.75; 17 -6.725,-3.25; 18 -6.725,-3.75; 19 -6.725,-4.25; 20 -6.725,-4.75; 41 6.725,-4.75; 42 6.725,-4.25; 43 6.725,-3.75; 44 6.725,-3.25; 45 6.725,-2.75; 46 6.725,-2.25; 47 6.725,-1.75; 48 6.725,-1.25; 49 6.725,-0.75; 50 6.725,-0.25; 51 6.725,0.25; 52 6.725,0.75; 53 6.725,1.25; 54 6.725,1.75; 55 6.725,2.25; 56 6.725,2.75; 57 6.725,3.25; 58 6.725,3.75; 59 6.725,4.25; 60 6.725,4.75 | smd 0.3 x 1.2: 21 -4.75,-6.725; 22 -4.25,-6.725; 23 -3.75,-6.725; 24 -3.25,-6.725; 25 -2.75,-6.725; 26 -2.25,-6.725; 27 -1.75,-6.725; 28 -1.25,-6.725; 29 -0.75,-6.725; 30 -0.25,-6.725; 31 0.25,-6.725; 32 0.75,-6.725; 33 1.25,-6.725; 34 1.75,-6.725; 35 2.25,-6.725; 36 2.75,-6.725; 37 3.25,-6.725; 38 3.75,-6.725; 39 4.25,-6.725; 40 4.75,-6.725; 61 4.75,6.725; 62 4.25,6.725; 63 3.75,6.725; 64 3.25,6.725; 65 2.75,6.725; 66 2.25,6.725; 67 1.75,6.725; 68 1.25,6.725; 69 0.75,6.725; 70 0.25,6.725; 71 -0.25,6.725; 72 -0.75,6.725; 73 -1.25,6.725; 74 -1.75,6.725; 75 -2.25,6.725; 76 -2.75,6.725; 77 -3.25,6.725; 78 -3.75,6.725; 79 -4.25,6.725; 80 -4.75,6.725
SOT223 = smd 1.5 x 2: 1 -2.3,-3.15; 2 0,-3.15; 3 2.3,-3.15 | smd 3.8 x 2: 4 0,3.15
SO16 = smd 0.66 x 2.032: 1 -4.445,-3.073; 2 -3.175,-3.073; 3 -1.905,-3.073; 4 -0.635,-3.073; 5 0.635,-3.073; 6 1.905,-3.073; 7 3.175,-3.073; 8 4.445,-3.073; 9 4.445,3.073; 10 3.175,3.073; 11 1.905,3.073; 12 0.635,3.073; 13 -0.635,3.073; 14 -1.905,3.073; 15 -3.175,3.073; 16 -4.445,3.073
2X03SMD = smd 1.016 x 3.302: 1 -1.27,-3.81; 2 -1.27,1.27; 3 1.27,-3.81; 4 1.27,1.27; 5 3.81,-3.81; 6 3.81,1.27
1X03SMD = smd 1.016 x 3.302: 1 -1.27,1.27; 2 1.27,-1.27; 3 3.81,1.27
1X02SMD = smd 1.016 x 3.302: 1 -1.27,1.27; 2 1.27,-1.27
2X10 = drill 1.016 octagon: 1 -11.43,-1.27; 2 -11.43,1.27; 3 -8.89,-1.27; 4 -8.89,1.27; 5 -6.35,-1.27; 6 -6.35,1.27; 7 -3.81,-1.27; 8 -3.81,1.27; 9 -1.27,-1.27; 10 -1.27,1.27; 11 1.27,-1.27; 12 1.27,1.27; 13 3.81,-1.27; 14 3.81,1.27; 15 6.35,-1.27; 16 6.35,1.27; 17 8.89,-1.27; 18 8.89,1.27; 19 11.43,-1.27; 20 11.43,1.27
0402 = smd 0.7 x 0.9: 1 -0.65,0; 2 0.65,0
CHIP-LED0805 = smd 1.2 x 1.2: A 0,-1.05; C 0,1.05
SM49 = smd 5.08 x 1.778: 1 -4.826,0; 2 4.826,0
R0805 = smd 1.3 x 1.5: 1 -0.85,0; 2 0.85,0
EXBS8V = smd 0.75 x 1.1: 1 -1.905,-1.07; 2 -0.635,-1.07; 3 0.635,-1.07; 4 1.905,-1.07; 5 1.905,1.07; 6 0.635,1.07; 7 -0.635,1.07; 8 -1.905,1.07
TASTER_93XX = smd 2.1 x 1.4: 1 -5,2.25; 2 5,2.25; 3 -5,-2.25; 4 5,-2.25
EDG-10 = drill 0.813 long: 1 -11.43,-3.81; 2 -8.89,-3.81; 3 -6.35,-3.81; 4 -3.81,-3.81; 5 -1.27,-3.81; 6 1.27,-3.81; 7 3.81,-3.81; 8 6.35,-3.81; 9 8.89,-3.81; 10 11.43,-3.81; 11 11.43,3.81; 12 8.89,3.81; 13 6.35,3.81; 14 3.81,3.81; 15 1.27,3.81; 16 -1.27,3.81; 17 -3.81,3.81; 18 -6.35,3.81; 19 -8.89,3.81; 20 -11.43,3.81
SOT23-BEC = smd 1 x 1.4: B -0.95,-1.1; C 0,1.1; E 0.95,-1.1
ASE = smd 0.9 x 0.65: 1 -1.05,-0.825; 2 1.05,-0.825; 3 1.05,0.825; 4 -1.05,0.825
LQFP48 = smd 1.5 x 0.3: 1 -4.15,2.75; 2 -4.15,2.25; 3 -4.15,1.75; 4 -4.15,1.25; 5 -4.15,0.75; 6 -4.15,0.25; 7 -4.15,-0.25; 8 -4.15,-0.75; 9 -4.15,-1.25; 10 -4.15,-1.75; 11 -4.15,-2.25; 12 -4.15,-2.75; 25 4.15,-2.75; 26 4.15,-2.25; 27 4.15,-1.75; 28 4.15,-1.25; 29 4.15,-0.75; 30 4.15,-0.25; 31 4.15,0.25; 32 4.15,0.75; 33 4.15,1.25; 34 4.15,1.75; 35 4.15,2.25; 36 4.15,2.75 | smd 0.3 x 1.5: 13 -2.75,-4.15; 14 -2.25,-4.15; 15 -1.75,-4.15; 16 -1.25,-4.15; 17 -0.75,-4.15; 18 -0.25,-4.15; 19 0.25,-4.15; 20 0.75,-4.15; 21 1.25,-4.15; 22 1.75,-4.15; 23 2.25,-4.15; 24 2.75,-4.15; 37 2.75,4.15; 38 2.25,4.15; 39 1.75,4.15; 40 1.25,4.15; 41 0.75,4.15; 42 0.25,4.15; 43 -0.25,4.15; 44 -0.75,4.15; 45 -1.25,4.15; 46 -1.75,4.15; 47 -2.25,4.15; 48 -2.75,4.15
3,2 = hole 3.2: 0,0
J1 = drill 0.9 pad 1.3: 1 4.445,2.54; 2 3.175,0; 3 1.905,2.54; 4 0.635,0; 5 -0.635,2.54; 6 -1.905,0; 7 -3.175,2.54; 8 -4.445,0 | drill 1 pad 1.422: 9 5.465,7.37; 10 2.925,7.37; 11 -2.925,7.37; 12 -5.465,7.37 | drill 1.6 pad 2.184: M1 -7.875,-3.3; M2 7.875,-3.3 | hole 3.3: 5.715,-6.35; -5.715,-6.35
UX60-MB-5ST = smd 2 x 0.5: 1 2.25,1.6; 2 2.25,0.8; 3 2.25,0; 4 2.25,-0.8; 5 2.25,-1.6 | smd 2.2 x 2.5: M1 -3.3,-4.2; M2 -3.3,4.2; M3 2,4.2; M4 2,-4.2 | hole 0.9: 0,-1.75; 0,1.75
733980-62 = drill 1 pad 2.5 long: 1 0,8.57; 2 0,2.42; 3 5,5.57
85-32004-10X = drill 0.92 pad 1.27: 1 4.71,-1.25; 2 4.71,1.25; 3 2.71,1.25; 4 2.71,-1.25 | drill 2.3 pad 3: M1 0,6.02; M2 0,-6.02

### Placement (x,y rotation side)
C1  39.41,32.49 270 top
C4  25.99,63.82 270 top
C5  25.94,47.87 90 top
C6  23.94,63.86 90 top
C7  11.43,69.85 0 top
C8  12.7,90.17 180 top
C9  16.51,93.98 0 top
C10  13.97,66.04 0 top
C11  31.85,53.67 180 top
C12  54.61,14.05 90 top
C13  57.46,13.4 270 top
C14  50.45,9.92 90 top
C15  45.67,10.06 90 top
C16  not placed on the board
C17  not placed on the board
C18  not placed on the board
C19  not placed on the board
C20  24.4,-3.1 270 top
C21  not placed on the board
C22  19.52,8.1 0 top
C23  40.91,-1.32 90 top
C24  not placed on the board
C25  not placed on the board
C26  13.67,15.88 90 top
C27  22.65,15.93 90 top
C28  33.25,62.82 0 top
C29  24.38,52.98 90 top
C30  28.75,63.83 270 top
C31  24.79,67.93 0 top
D1  not placed on the board
D2  not placed on the board
D3  not placed on the board
D4  49.1,-1.08 0 top
DMX1IN  151.13,83.82 270 top
DMX1OUT  154.94,83.82 90 top
DMX2OUT  154.94,67.31 90 top
DMX3OUT  154.94,55.88 90 top
DMX4OUT  154.94,44.45 90 top
IC1  30.04,30.2 0 bottom
IC6  32.05,-1.67 0 top
IC7  not placed on the board
IC8  18.23,15.98 0 top
IC10  115.85,85.85 90 top
IC11  115.5,68.5 90 top
IC12  118.5,55 90 top
IC13  118.35,41.8 90 top
J3  151.13,67.31 270 top
J5  151.13,55.88 270 top
J7  151.13,44.45 270 top
JP1  32.37,30.65 270 top
JP2  40.64,18.24 270 top
JP3  28.36,15.68 90 top
JP4  17.8,51.21 90 top
JP5  not placed on the board
JP6  not placed on the board
JP7  not placed on the board
JP8  52.85,33.19 270 top
L1  not placed on the board
LED1  24.13,99.06 270 top
LED2  not placed on the board
LED3  not placed on the board
LED4  6.06,18.19 90 top
LED5  147.32,77.47 90 top
LED6  146.05,60.96 90 top
LED7  146.05,50.8 90 top
LED8  146.05,35.56 90 top
Q1  38.81,17.49 90 top
Q2  47.08,21.88 90 top
R1  152.4,90.17 0 top
R2  39.41,29.06 90 top
R3  29.13,67.94 0 top
R4  32.59,66.88 270 top
R5  21.97,63.88 270 top
R6  20.32,77.47 0 top
R7  20.32,82.55 0 top
R8  20.32,85.09 180 top
R9  20.42,74.33 0 top
R10  25.24,95.35 90 top
R11  19.05,99.06 180 top
R12  38.34,54.99 0 top
R13  not placed on the board
R14  16.51,90.17 0 top
R15  11.43,93.98 0 top
R16  16.51,69.85 180 top
R17  8.89,66.04 0 top
R18  not placed on the board
R19  not placed on the board
R20  not placed on the board
R21  not placed on the board
R22  not placed on the board
R23  not placed on the board
R24  not placed on the board
R25  not placed on the board
R26  10.09,18.19 180 top
R27  40.48,62.95 0 top
R28  152.4,74.93 0 top
R29  153.67,60.96 0 top
R30  153.67,49.53 0 top
R31  26.22,44.37 180 top
R32  142.24,77.47 0 top
R33  142.24,60.96 0 top
R34  140.97,49.53 0 top
R35  140.97,35.56 0 top
RN1  48.35,39.07 270 top
RN2  47.58,26.11 270 top
S1  41.71,40.7 90 top
S2  37.4,70.79 270 top
SW1  6,33.25 270 top
T1  not placed on the board
U$1  31.75,55.91 180 top
U$2  30.55,54.79 180 top
U$3  [3,2]  5.08,95.25 0 top
X1  8.89,80.01 270 top
X2  not placed on the board
X3  2.77,11.33 270 top
X4  not placed on the board

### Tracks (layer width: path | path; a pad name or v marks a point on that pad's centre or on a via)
+3.3VA  (2 unrouted)
+3V3  (via drill 0.5)  (34 unrouted)
  Top 0.305: R3.1 27.4,67.94 27.4,62.85 28.75,62.85 C30.2 28.75,62.8 28.8,62.8 U$2.22 28.8,54.04 U$2.32 24.38,54.04 C29.2 22.1,53.98 22.1,47.7 25.37,44.45 R31.2 | R3.1 C31.2 | R3.1 28.3,67.93 28.3,69.55 32.59,69.55 R4.1 | U$2.48 33.25,50.64 33.25,50.45 | 33.25,50.45 33.25,42.35 v33.6,42.35 | R2.1 39.4,27.71 39.35,27.71 39.35,24.15 v36.2,24.15 | R27.2 41.33,57.37 43.7,55 43.7,52.95 v42.2,51.45 41.4,50.65 33.45,50.65 33.25,50.45 | JP8.1 JP8.2 | v48.6,41 49.4,41 RN1.8 RN1.7 RN1.6 | IC8.4 13.67,19.13 C26.2 | C27.2 22.85,16.93 22.85,19.13
  Top 0.61: IC8.4 22.85,19.13 24.1,19.13 24.1,21.8 36.2,21.8 v36.2,24.15
  Bottom 0.305: IC1.56 25,32.95 28.85,30.1 28.85,25.7 | 28.85,25.7 24.5,25.7 24.5,25.95 IC1.42 | IC1.21 34.79,24.15 | 34.79,24.15 34.79,25.7 32.45,25.7 | 32.45,25.7 28.85,25.7 | v33.6,42.35 33.29,42.35 IC1.77 33.29,29.44 32.95,28.75 32.49,27.85 32.45,25.7 | v36.2,24.15 34.79,24.15 | JP8.1 49.08,44.62 48.9,44.8 | 48.9,44.8 v42.2,51.45 | v48.6,41 48.9,41.3 48.9,44.8
+5V  (6 unrouted)
BUTTON_RESERVE  (via drill 0.5)
  Top 0.305: S2.2 S2.1 | S2.2 39.65,62.97 R27.1 34.38,62.95 C28.2 | v29.55,34.6 30.75,33.4 32.05,33.4 33,34.35 33,39.95 35,41.95 35.05,49.55 42.05,49.55 45,52.5 45,63.55 42.75,65.8 42.7,65.8 S2.2
  Bottom 0.305: IC1.68 28.79,35.36 v29.55,34.6
DERE0  (via drill 0.5)  (2 unrouted)
  Top 0.305: v19.25,41.45 11.6,49.1 v4.5,49.1
  Bottom 0.305: IC1.61 25.21,37.9 21.45,37.9 19.25,40.1 v19.25,41.45 | v4.5,49.1 4.5,72.45 84.6,72.45
DERE1  (via drill 0.5)  (2 unrouted)
  Top 0.305: v20.55,41.6 12.15,50.05 v3.5,50.05
  Bottom 0.305: IC1.62 25.79,38.7 21.75,38.7 20.55,39.9 v20.55,41.6 | v3.5,50.05 3.5,73.15 83.9,73.15
DERE2  (via drill 0.5)  (2 unrouted)
  Top 0.305: v17.65,41.55 11.1,48.1 v2.4,48.1
  Bottom 0.305: IC1.63 26.29,35.55 24.9,35.55 23.6,36.85 21.15,36.85 17.65,40.35 v17.65,41.55 | v2.4,48.1 2.4,73.85 83.25,73.85
DERE3  (via drill 0.5)  (2 unrouted)
  Top 0.305: v22,41.5 12.3,51.15 v1.4,51.2
  Bottom 0.305: IC1.64 26.79,39.35 23,39.35 21.95,40.4 v22,41.5 | v1.4,51.2 1.4,74.5 82.3,74.5
DIP1_DMX1_IN/OUT  (via drill 0.5)
  Top 0.305: v23.2,35.7 20.85,35.7 19.45,37.1 17.7,37.1 10.12,44.68 SW1.20
  Bottom 0.305: IC1.60 23.2,34.95 v23.2,35.7
DIP2_DMX2_IN/OUT  (via drill 0.5)
  Top 0.305: v24.55,34.45 20.55,34.45 19,36 17.05,36 10.9,42.15 9.32,42.15 SW1.19
  Bottom 0.305: IC1.59 v24.55,34.45
DIP3_DMX3_IN/OUT  (via drill 0.5)
  Top 0.305: v19.7,33.95 18.7,34.95 15.45,34.95 10.8,39.6 SW1.18
  Bottom 0.305: IC1.58 v19.7,33.95
DIP4_DMX4_IN/OUT  (via drill 0.5)
  Top 0.305: v17.8,33.95 14.2,33.95 11.09,37.06 SW1.17
  Bottom 0.305: 23.4,32.45 IC1.55 19.65,32.45 18.15,33.95 v17.8,33.95
DIP5  (via drill 0.5)
  Top 0.305: v24.55,31.95 19.2,31.95 18.2,32.95 13.1,32.95 11.53,34.52 SW1.16
  Bottom 0.305: IC1.54 v24.55,31.95
DIP6  (via drill 0.5)
  Top 0.305: v17.85,31.95 9.34,31.95 arc-90 SW1.15
  Bottom 0.305: IC1.53 18.35,31.45 v17.85,31.95
DIP7  (via drill 0.5)
  Top 0.305: v17.85,30.4 10.27,30.4 SW1.14
  Bottom 0.305: IC1.52 18.4,30.95 v17.85,30.4
DIP8  (via drill 0.5)
  Top 0.305: v24.55,30.45 19.25,30.45 18.25,29.45 13.2,29.45 10.65,26.9 SW1.13
  Bottom 0.305: IC1.51 v24.55,30.45
DIP9  (via drill 0.5)
  Top 0.305: v23.35,24.7 22.1,24.7 18.25,28.55 14,28.55 SW1.12
  Bottom 0.305: IC1.41 23.35,25.41 v23.35,24.7
DIP10_NETMASK  (via drill 0.5)
  Top 0.305: v25.4,40.15 17.1,40.15 10.5,46.75 7.3,46.75 7.35,23.2 8.75,21.85 9.28,21.85 SW1.11
  Bottom 0.305: IC1.65 27.3,36.94 27.3,40.15 v25.4,40.15
ENET_CRS  (via drill 0.5)
  Top 0.305: U$2.40 29.3,48.1 28.75,47.55 28.75,43.15 v27.9,42.3
  Bottom 0.305: v27.9,42.3 31.29,42.3 IC1.73
ENET_MDC  (via drill 0.5)
  Top 0.305: v27.95,54.75 27.74,54.54 U$2.31
  Bottom 0.305: IC1.50 19.1,29.95 19.1,28.85 16.6,28.85 16.6,54.6 27.95,54.6 v27.95,54.75
ENET_MDIO
  Top 0.305: U$2.30 16.55,55.04 arc90 JP4.3
ENET_REF_CLK  (via drill 0.5)  (1 unrouted)
  Top 0.305: v28.65,53.04 U$2.34
  Bottom 0.305: IC1.69 29.29,39.41 22.7,46 22.7,53.04 v28.65,53.04
ENET_RX_ER  (via drill 0.5)
  Top 0.305: v29.3,41.25 29.3,46.85 29.8,47.35 U$2.41
  Bottom 0.305: IC1.70 29.79,40.69 v29.3,41.25
ENET_RXD0  (via drill 0.5)
  Top 0.305: v30.5,46.05 30.8,46.05 U$2.43
  Bottom 0.305: IC1.72 30.79,46.05 v30.5,46.05
ENET_RXD1  (via drill 0.5)
  Top 0.305: v31.3,34.75 U$2.44
  Bottom 0.305: IC1.71 30.29,35.76 v31.3,34.75
ENET_TX_EN  (via drill 0.5)
  Top 0.305: v37.5,52.1 37.06,52.54 U$2.2
  Bottom 0.305: IC1.74 31.79,46.39 v37.5,52.1
ENET_TXD0  (via drill 0.5)
  Top 0.305: v41.8,53.05 34.81,53.05 U$2.3
  Bottom 0.305: IC1.76 32.79,44.04 v41.8,53.05
ENET_TXD1  (via drill 0.5)
  Top 0.305: v41.75,54.5 40.79,53.54 U$2.4
  Bottom 0.305: IC1.75 32.29,45.04 v41.75,54.5
GND  (via drill 0.5)  (54 unrouted)
  Top 0.305: v33.3,24.7 v33.29,24.7 | v33.29,24.7 v28.8,24.7 | v25.95,26.45 v25.95,33.45 | v31.3,27.8 v33.75,27.8 33.75,26.95 JP1.6 33.64,25.05 v33.29,24.7 | U$2.47 v32.8,52.05 | v27.6,52.05 v27.6,52.04 U$2.36 | U$2.35 U$2.36 | v32.3,57.65 U$2.15 32.3,61.63 C28.1 32.3,62.87 32.3,64.3 33.66,64.3 S2.4 S2.3 | v30.3,57.65 U$2.19 | C4.1 v25.99,66.25 v26,66.25 | v28.75,66.25 C30.1 | R5.1 21.97,66.25 v21.95,66.25 | C6.2 v23.94,66.25 v23.9,66.25 | v23.95,66.25 23.95,67.93 C31.1 | U$2.36 26.4,51.98 C29.1 24.38,46.87 C5.1 27.4,46.87 v27.4,46.85 | C1.1 39.46,33.54 S1.1 S1.2 | RN2.4 46.51,24.09 50.35,20.25 52.91,20.25 JP8.20 | RN1.5 50.88,35.7 52.8,35.7 54.04,34.46 JP8.10 | C27.1 15.93,14.93 IC8.1
  Bottom 0.305: IC1.24 v33.29,24.7 v33.3,24.7 | v28.8,24.7 IC1.33 | IC1.43 v25.95,26.45 | v25.95,33.45 IC1.57 | IC1.66 27.79,35.7 v31.3,27.8 | v33.75,27.8 IC1.78 | v32.8,52.05 v27.6,52.05 | v32.3,57.65 31.55,57.65 | 31.55,57.65 v30.3,57.65 | v21.95,66.25 v23.9,66.25 v23.95,66.25 v26,66.25 v28.75,66.25 31.55,66.25 31.55,57.65 | v27.4,46.85 27.45,46.85 27.45,46.7
  pour Bottom: 0.55,99.45 57.3,99.75 49.05,52.75 80.9,14.85 66.8,1.75 -5.4,1.75 -20.5,16.85 -20.5,78.4
  pour Top: -1.8,-0.95 -4.6,-0.95 -12.6,7.05 -13.55,14.3 -5.45,22.4 66.8,22.35 67.95,21.2 67.95,1.85 61.55,-4.55 2,-4.55 -1.75,-0.8
LED_ACT  (2 unrouted)
LED_DMX1_RECEIV_DATA  (1 unrouted)
LED_DMX2_RECEIV_DATA  (1 unrouted)
LED_DMX3_RECEIV_DATA  (1 unrouted)
LED_DMX4_RECEIV_DATA  (1 unrouted)
LED_LINK  (2 unrouted)
LED_SPEED  (2 unrouted)
MISO  (via drill 0.5)
  Top 0.305: v27.7,27.95 28.56,27.95 JP1.5
  Bottom 0.305: IC1.46 v27.7,27.95
MOSI  (via drill 0.5)
  Top 0.305: JP1.4 36,29.38 36,25.55 35.95,25.55 33.8,23.4 26.3,23.4 24.75,24.95 v24.75,27.2
  Bottom 0.305: v24.75,27.2 24.5,27.45 IC1.45
N$1  (3 unrouted)
N$2  (3 unrouted)
N$4  (1 unrouted)
N$5  (1 unrouted)
N$6  (1 unrouted)
N$7
  Top 0.305: 25.8,52.5 25.8,52.05 26.1,52.05 26.1,52.5 26.7,52.5 26.7,52.05 26.95,52.05 26.95,52.5
N$8  (1 unrouted)
N$9  (1 unrouted)
N$10
  Top 0.305: U$2.7 38.04,55.04 R12.1
N$11  (2 unrouted)
N$12  (2 unrouted)
N$13  (2 unrouted)
N$14
  Top 0.305: U$2.21 29.3,61.6 30.1,61.6 30.05,67.94 R3.2
N$15
  Top 0.305: R4.2 30.75,66.03 30.75,61.05 29.8,61.05 U$2.20
N$16  (2 unrouted)
N$17  (2 unrouted)
  Top 0.305: U$2.23 28.3,61.6 26,61.6 | 26,61.6 C4.2 | C6.1 23.94,61.6 26,61.6 | U$2.37 27.8,48.85 27.14,48.85 C5.2
N$18
  Top 0.305: U$2.24 25.31,58.94 21.95,62.3 21.95,63.01 R5.2
N$19
  Top 0.305: U$2.39 28.8,48.7 28.25,48.15 28.25,44.4 R31.1
N$20  (2 unrouted)
N$21  (1 unrouted)
N$22  (via drill 0.5)
  Top 0.305: JP2.1 36.85,19.49 v36.85,18.25 36.85,16.99 JP2.3 JP2.5
  Bottom 0.305: IC1.22 34.29,20.81 v36.85,18.25
N$23  (via drill 0.5)
  Top 0.305: JP3.5 32.2,19.46 v32.2,18.2 32.2,16.98 JP3.3 JP3.1
  Bottom 0.305: IC1.23 33.79,19.79 v32.2,18.2
N$24  (2 unrouted)
N$25  (via drill 0.5)
  Top 0.305: v15.4,52.5 19.07,52.5 JP4.2
  Bottom 0.305: IC1.49 19.9,29.45 19.9,28 15.55,28 15.55,48.15 13.8,48.15 13.8,52.45 15.4,52.45 v15.4,52.5
N$26  (1 unrouted)
N$27  (1 unrouted)
N$28  (2 unrouted)
N$29  (1 unrouted)
N$30  (4 unrouted)
N$31  (2 unrouted)
N$32  (1 unrouted)
N$33  (1 unrouted)
N$35  (2 unrouted)
N$36  (3 unrouted)
N$37  (3 unrouted)
N$38  (3 unrouted)
N$39  (3 unrouted)
N$40  (3 unrouted)
N$41  (3 unrouted)
N$42
  Top 0.305: RN2.5 49.13,24.2 JP8.19
N$43
  Top 0.305: RN2.6 50.01,25.48 JP8.17
N$44  (1 unrouted)
N$45  (1 unrouted)
RD+  (2 unrouted)
RD-  (2 unrouted)
RST  (via drill 0.5)  (1 unrouted)
  Top 0.305: v34.85,30.65 29.83,30.65 JP1.1 28.56,33.09 27.05,34.6 27.05,40.05 21.3,45.8 21.3,53.75 21.25,53.8 14.2,53.8 14.15,53.85 14.15,56.2 19.65,56.2 19.65,55.54 U$2.29 | C1.2 R2.2 39.41,29.95 v41.15,29.95 43.96,29.99 S1.3 S1.4
  Bottom 0.305: v34.85,30.65 34.85,28.45 IC1.14 47.35,28.45 48.95,26.85 49.12,26.85 JP8.15
RTCK
  Top 0.305: RN2.8 48.65,28.99 JP8.11
RXD0  (via drill 0.5)  (1 unrouted)
  Top 0.305: v41.85,46.3 61.35,65.8 82.6,65.8
  Bottom 0.305: IC1.80 34.79,39.24 v41.85,46.3
RXD1  (1 unrouted)
  Bottom 0.305: IC1.48 20.55,28.95 20.55,27.05 14.45,27.05 14.45,46.7 12.6,46.7 12.6,67.65 84.05,67.65 84.05,67.6
RXD2  (1 unrouted)
  Bottom 0.305: IC1.40 11.9,23.48 11.9,20.4 7.7,20.4 7.7,69.55 84.2,69.55 84.2,69.8
RXD3  (1 unrouted)
  Bottom 0.305: IC1.38 26.29,22.19 25.15,21.05 13.2,21.05 13.2,19.25 6.15,19.25 6.15,70.9 83.1,70.9 83.1,71
TCK/SWDCLK
  Top 0.305: RN1.4 49.98,34.46 JP8.9
  Bottom 0.305: IC1.5 42.55,32.95 44.05,34.45 46.92,34.45 JP8.9
TD+  (2 unrouted)
TD-  (2 unrouted)
TDI  (via drill 0.5)
  Top 0.305: RN1.2 47.28,39.6 v46.5,39.7
  Bottom 0.305: IC1.2 38.7,34.45 43.85,39.6 46.45,39.6 v46.5,39.7 46.87,39.6 JP8.5
TDO/SWO  (via drill 0.5)
  Top 0.305: RN2.7 48.95,26.75 JP8.13 | v41.75,40.7 41.75,32.2 v42.6,31.35
  Bottom 0.305: IC1.1 36.77,35.72 v41.75,40.7 | v42.6,31.35 49.66,31.3 JP8.13
TMS/SWDIO  (via drill 0.5)
  Top 0.305: v46.45,38.45 RN1.3
  Bottom 0.305: IC1.3 40.5,33.95 43.6,37.05 46.45,37.05 | JP8.7 46.88,37.05 46.45,37.05 | 46.45,37.05 v46.45,38.45
TRST_N  (via drill 0.5)
  Top 0.305: v45.45,35.9 45.4,42.05 47.35,42.06 | 47.35,42.06 JP8.3 | RN1.1 47.28,42.06 47.35,42.06
  Bottom 0.305: IC1.4 41.65,33.45 44,35.8 45.35,35.8 v45.45,35.9
TXD0  (via drill 0.5)  (1 unrouted)
  Top 0.305: v42.85,48.8 60.85,66.8 83.8,66.8
  Bottom 0.305: IC1.79 34.29,40.24 v42.85,48.8
TXD1  (1 unrouted)
  Bottom 0.305: IC1.47 21.25,28.45 21.25,26.3 13.5,26.3 13.5,45.6 11.75,45.6 11.75,68.55 83.95,68.55
TXD2  (1 unrouted)
  Bottom 0.305: IC1.39 25.79,22.44 25.2,21.85 12.55,21.85 12.55,19.85 6.9,19.85 6.9,70.25 82.5,70.25 82.5,70.2
TXD3  (1 unrouted)
  Bottom 0.305: IC1.37 26.79,21.84 25.3,20.35 13.9,20.35 13.9,18.55 5.4,18.55 5.4,71.7 83.4,71.7 83.4,71.75
USB  (2 unrouted)
USB-MODE  (1 unrouted)
USB_D+  (2 unrouted)
USB_D-  (2 unrouted)
USB_PWRD  (1 unrouted)
USB_UP_LED  (1 unrouted)
VBUS  (1 unrouted)
VCC  (6 unrouted)
  Top 0.305: R26.1 11.34,17.79 X3.1
  Top 0.406: IC8.3 | 20.52,10.05 C22.2
  Top 1.27: X3.1 12.62,10.05 20.52,10.05 20.53,10.06 IC8.3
